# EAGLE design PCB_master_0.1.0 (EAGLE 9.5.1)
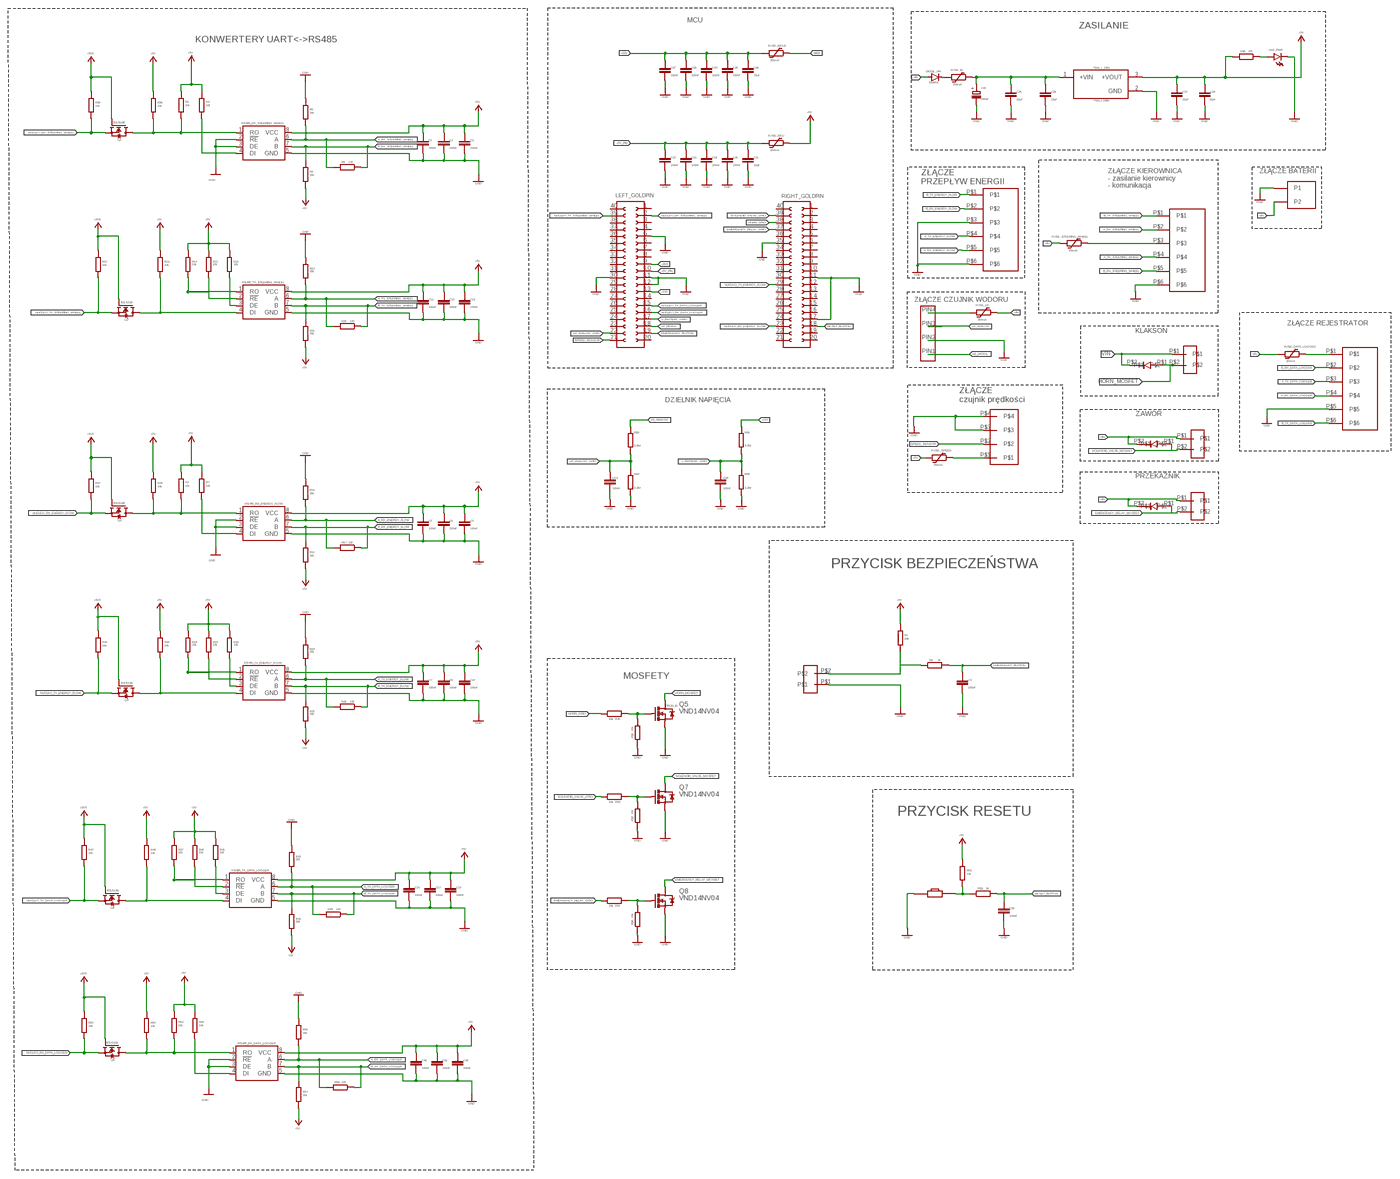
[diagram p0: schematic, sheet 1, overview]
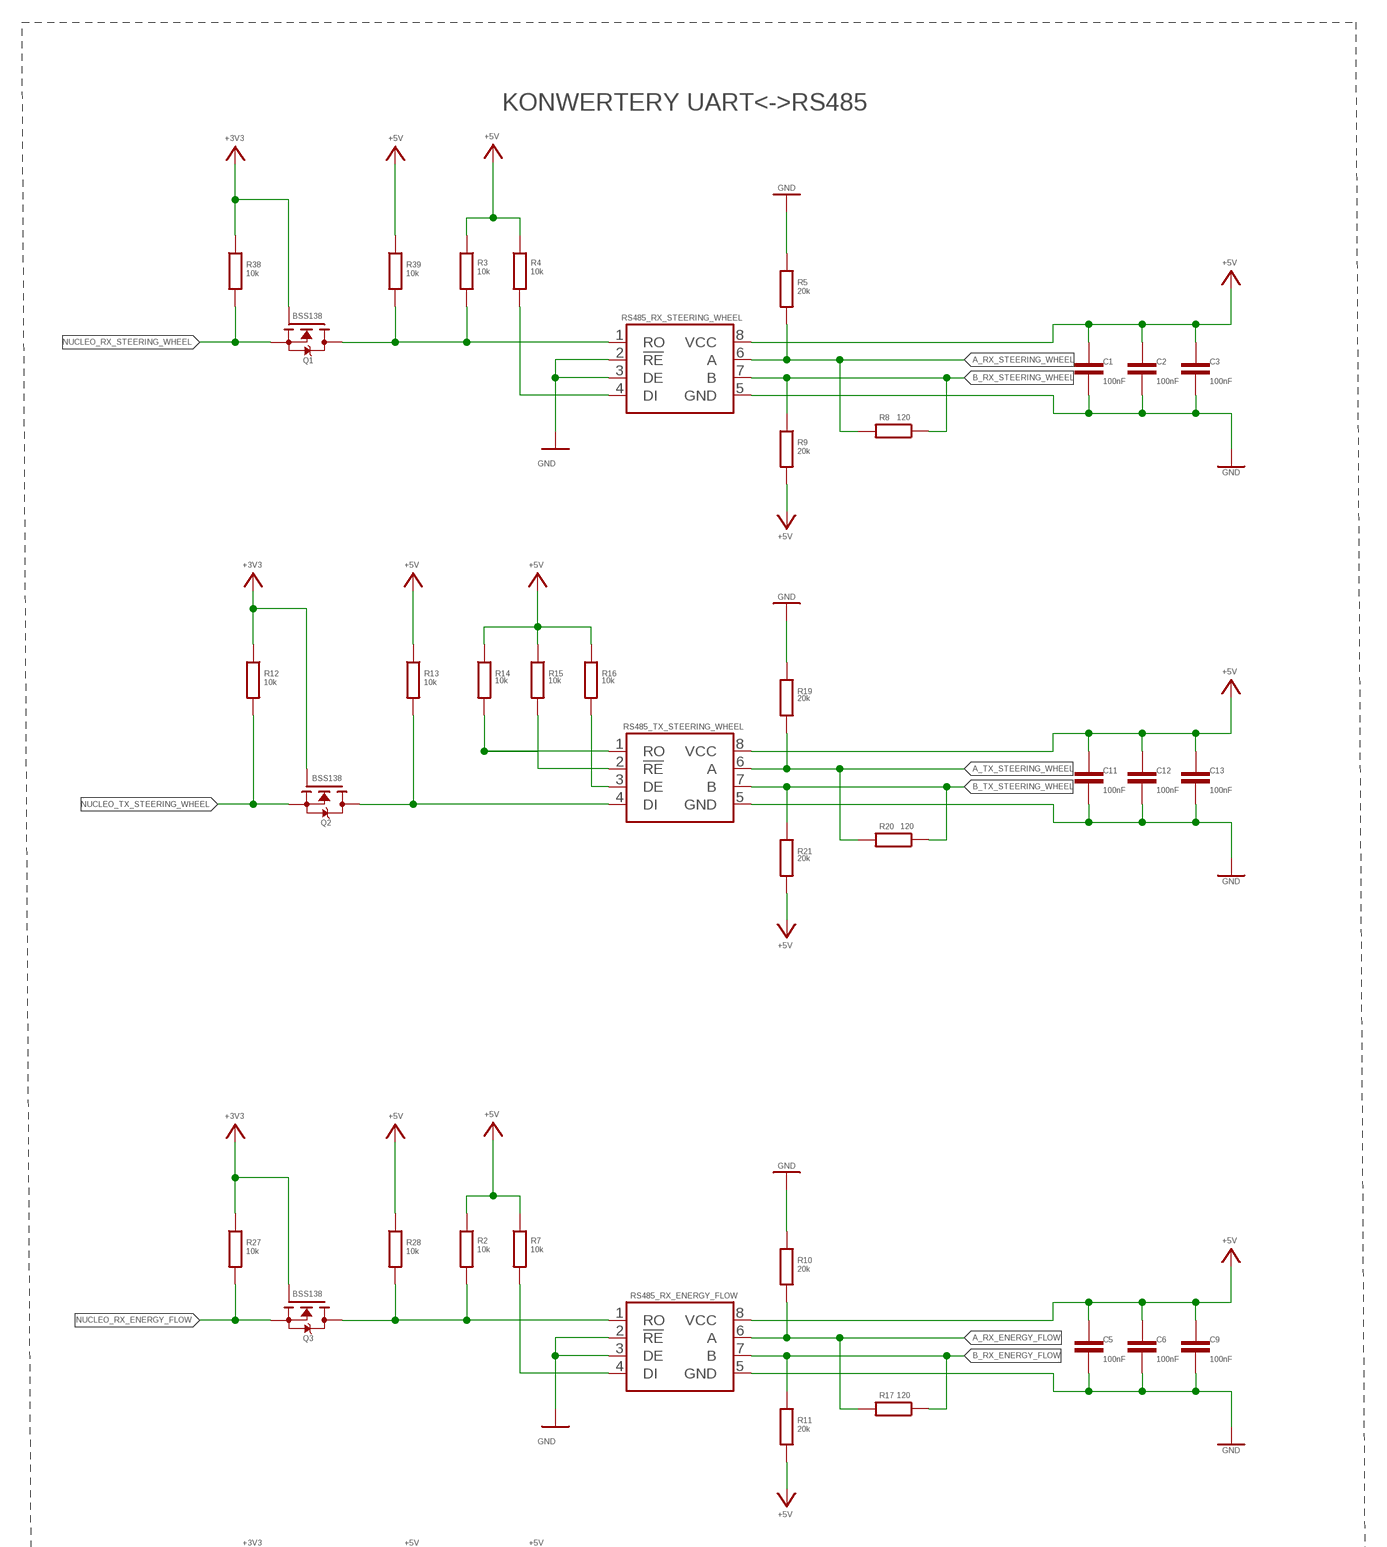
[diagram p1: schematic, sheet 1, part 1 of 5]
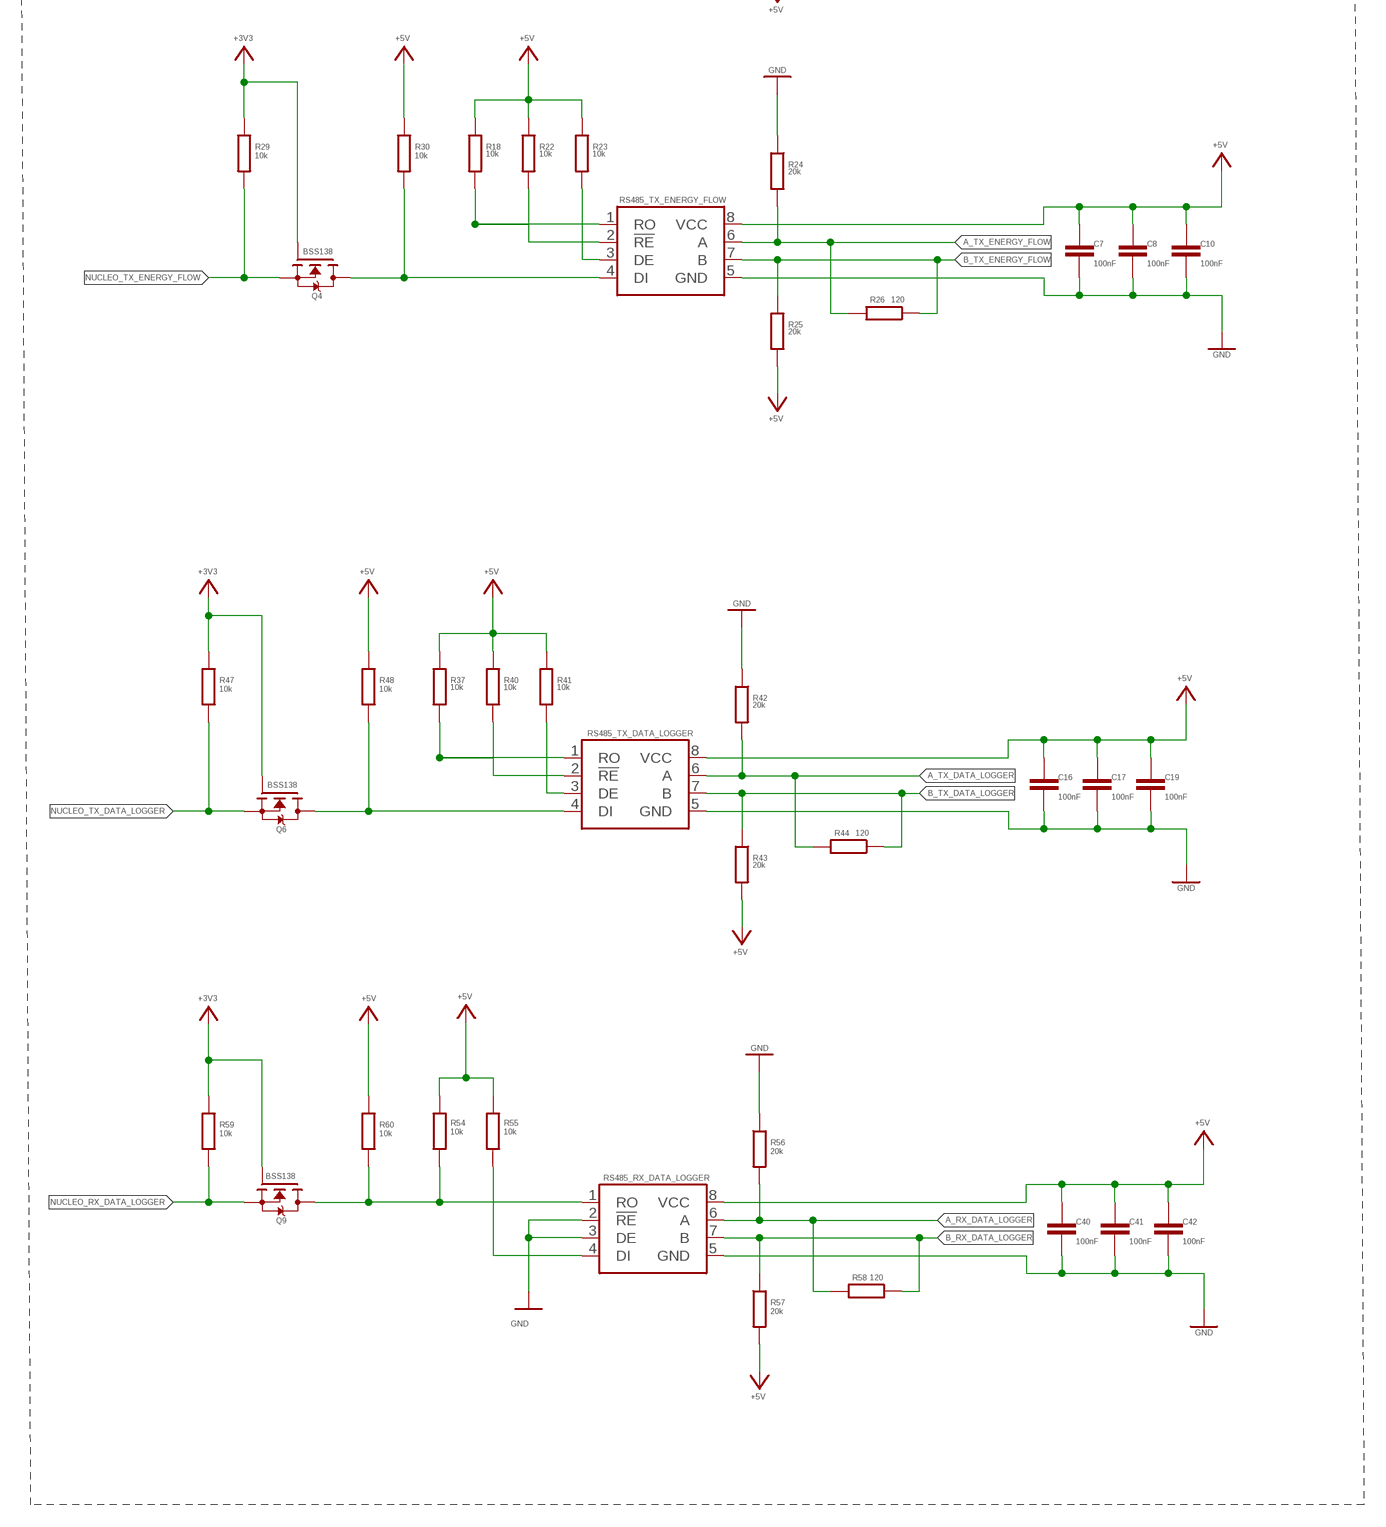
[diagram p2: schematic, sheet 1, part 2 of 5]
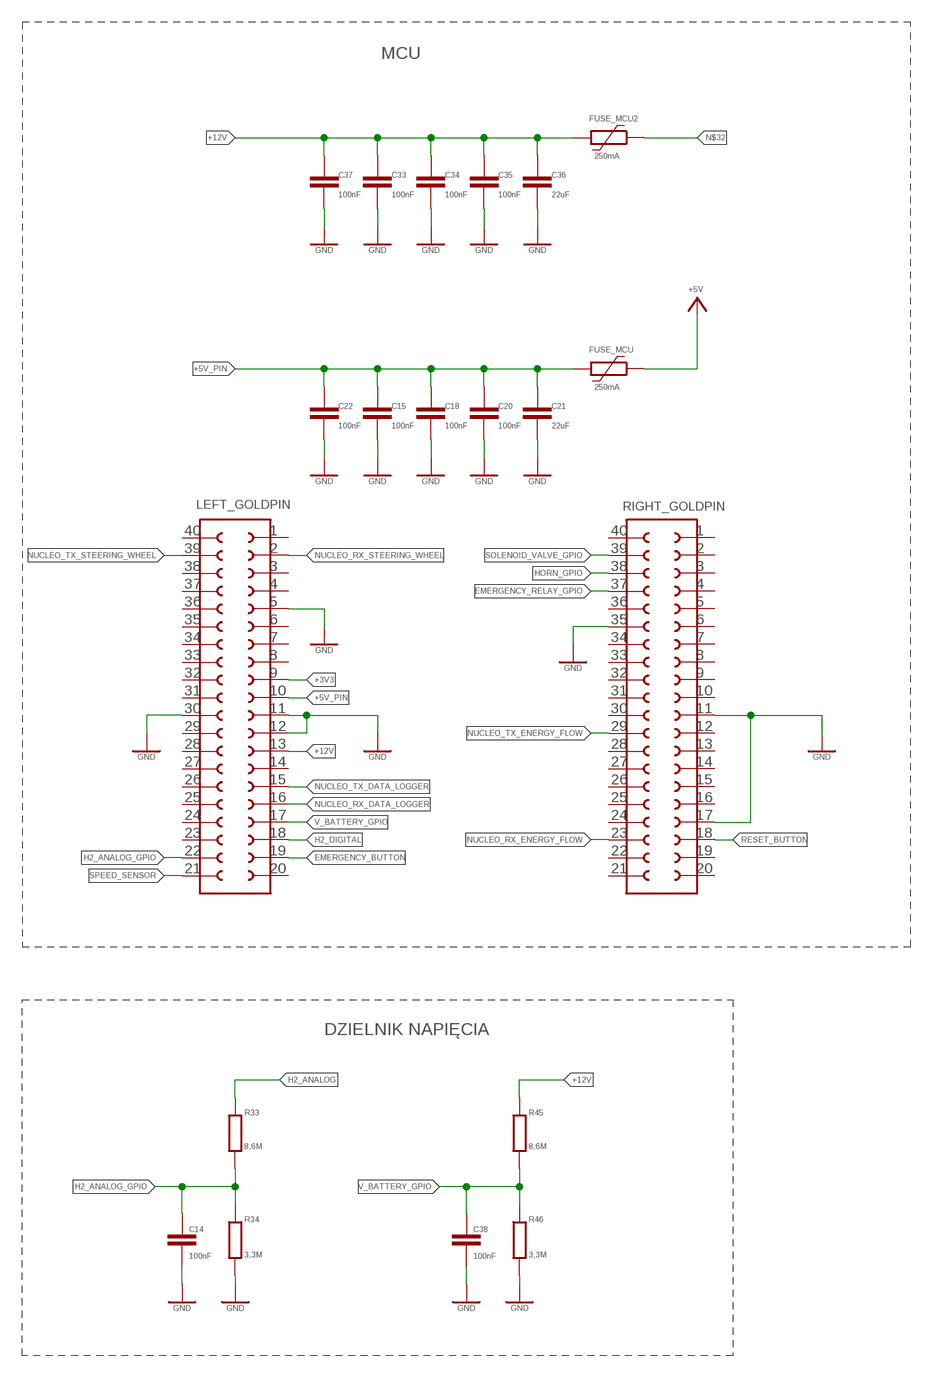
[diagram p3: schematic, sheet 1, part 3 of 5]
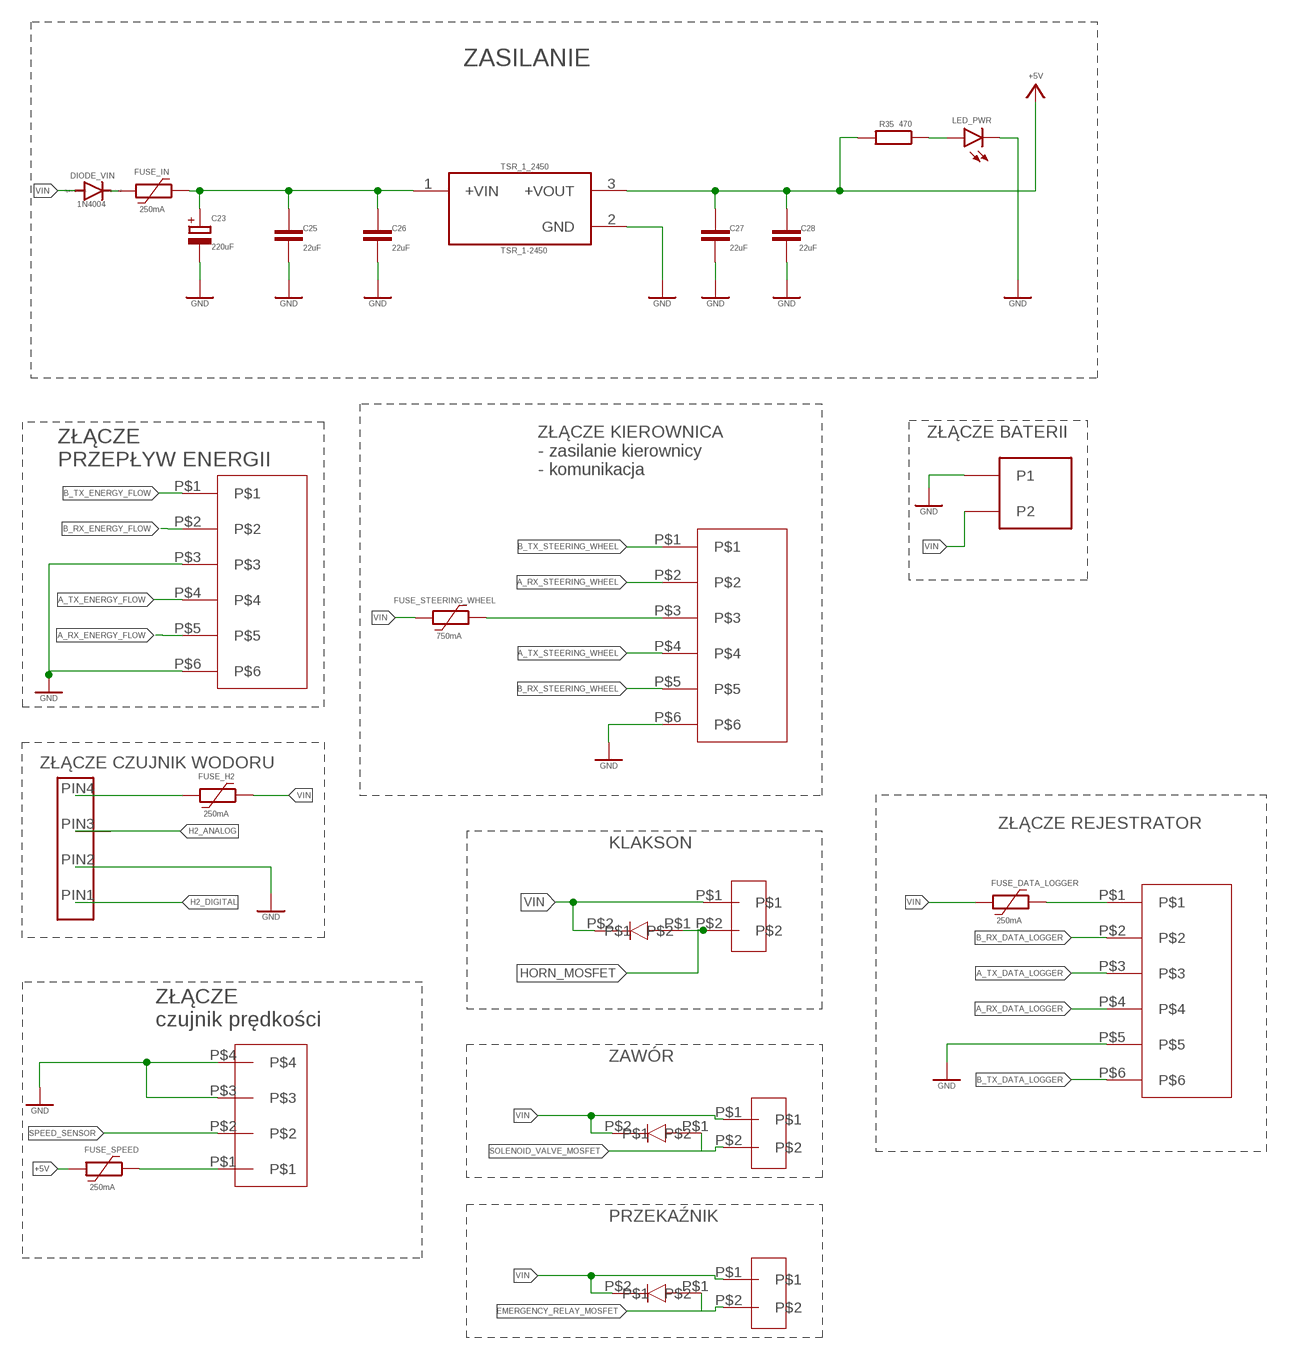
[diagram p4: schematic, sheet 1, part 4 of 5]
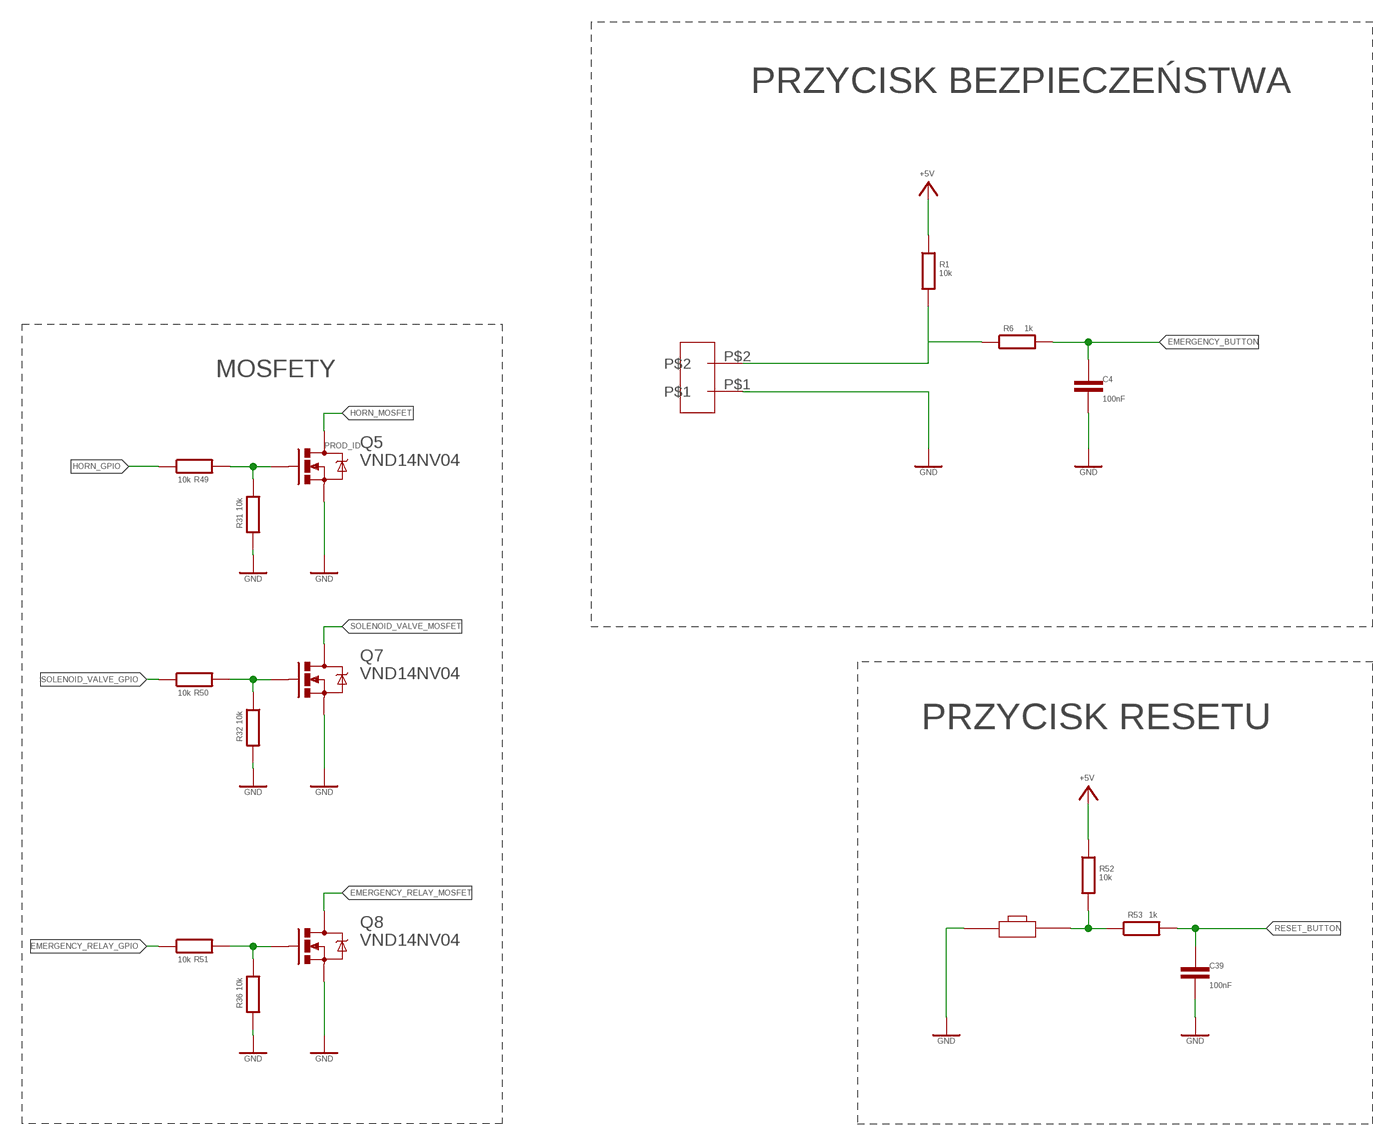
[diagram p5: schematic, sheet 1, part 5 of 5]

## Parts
C1  100nF  C-EUC1206  [C1206]
C2  100nF  C-EUC1206  [C1206]
C3  100nF  C-EUC1206  [C1206]
C4  100nF  C-EUC1206  [C1206]
C5  100nF  C-EUC1206  [C1206]
C6  100nF  C-EUC1206  [C1206]
C7  100nF  C-EUC1206  [C1206]
C8  100nF  C-EUC1206  [C1206]
C9  100nF  C-EUC1206  [C1206]
C10  100nF  C-EUC1206  [C1206]
C11  100nF  C-EUC1206  [C1206]
C12  100nF  C-EUC1206  [C1206]
C13  100nF  C-EUC1206  [C1206]
C14  100nF  C-EUC1206  [C1206]
C15  100nF  C-EUC1206  [C1206]
C16  100nF  C-EUC1206  [C1206]
C17  100nF  C-EUC1206  [C1206]
C18  100nF  C-EUC1206  [C1206]
C19  100nF  C-EUC1206  [C1206]
C20  100nF  C-EUC1206  [C1206]
C21  22uF  C-EUC1206  [C1206]
C22  100nF  C-EUC1206  [C1206]
C23  220uF  CPOL-EUUD-8X10  [UD-8X10_NICHICON]
C25  22uF  C-EUC1206  [C1206]
C26  22uF  C-EUC1206  [C1206]
C27  22uF  C-EUC1206  [C1206]
C28  22uF  C-EUC1206  [C1206]
C33  100nF  C-EUC1206  [C1206]
C34  100nF  C-EUC1206  [C1206]
C35  100nF  C-EUC1206  [C1206]
C36  22uF  C-EUC1206  [C1206]
C37  100nF  C-EUC1206  [C1206]
C38  100nF  C-EUC1206  [C1206]
C39  100nF  C-EUC1206  [C1206]
C40  100nF  C-EUC1206  [C1206]
C41  100nF  C-EUC1206  [C1206]
C42  100nF  C-EUC1206  [C1206]
DIODE_VIN  1N4004  [DO41-10]
FUSE_DATA_LOGGER  250mA  1206L012  [1206L]
FUSE_H2  250mA  1206L012  [1206L]
FUSE_IN  250mA  1206L012  [1206L]
FUSE_MCU  250mA  1206L012  [1206L]
FUSE_MCU2  250mA  1206L012  [1206L]
FUSE_SPEED  250mA  1206L012  [1206L]
FUSE_STEERING_WHEEL  750mA  2920L030  [2920L]
LED_PWR  LEDSMT1206  [1206]
LEFT_GOLDPIN  61304021821  [61304021821]
Q1  BSS138  [SOT23]
Q2  BSS138  [SOT23]
Q3  BSS138  [SOT23]
Q4  BSS138  [SOT23]
Q5  VND14NV04  MOSFET-NCHANNELFDD8780  [DPAK]
Q6  BSS138  [SOT23]
Q7  VND14NV04  MOSFET-NCHANNELFDD8780  [DPAK]
Q8  VND14NV04  MOSFET-NCHANNELFDD8780  [DPAK]
Q9  BSS138  [SOT23]
R1  10k  R-EU_R1206  [R1206]
R2  10k  R-EU_R1206  [R1206]
R3  10k  R-EU_R1206  [R1206]
R4  10k  R-EU_R1206  [R1206]
R5  20k  R-EU_R1206  [R1206]
R6  1k  R-EU_R1206  [R1206]
R7  10k  R-EU_R1206  [R1206]
R8  120  R-EU_R1206  [R1206]
R9  20k  R-EU_R1206  [R1206]
R10  20k  R-EU_R1206  [R1206]
R11  20k  R-EU_R1206  [R1206]
R12  10k  R-EU_R1206  [R1206]
R13  10k  R-EU_R1206  [R1206]
R14  10k  R-EU_R1206  [R1206]
R15  10k  R-EU_R1206  [R1206]
R16  10k  R-EU_R1206  [R1206]
R17  120  R-EU_R1206  [R1206]
R18  10k  R-EU_R1206  [R1206]
R19  20k  R-EU_R1206  [R1206]
R20  120  R-EU_R1206  [R1206]
R21  20k  R-EU_R1206  [R1206]
R22  10k  R-EU_R1206  [R1206]
R23  10k  R-EU_R1206  [R1206]
R24  20k  R-EU_R1206  [R1206]
R25  20k  R-EU_R1206  [R1206]
R26  120  R-EU_R1206  [R1206]
R27  10k  R-EU_R1206  [R1206]
R28  10k  R-EU_R1206  [R1206]
R29  10k  R-EU_R1206  [R1206]
R30  10k  R-EU_R1206  [R1206]
R31  10k  R-EU_R1206  [R1206]
R32  10k  R-EU_R1206  [R1206]
R33  8,2M  R-EU_M1206  [M1206]
R34  3,3M  R-EU_M1206  [M1206]
R35  470  R-EU_R1206  [R1206]
R36  10k  R-EU_R1206  [R1206]
R37  10k  R-EU_R1206  [R1206]
R38  10k  R-EU_R1206  [R1206]
R39  10k  R-EU_R1206  [R1206]
R40  10k  R-EU_R1206  [R1206]
R41  10k  R-EU_R1206  [R1206]
R42  20k  R-EU_R1206  [R1206]
R43  20k  R-EU_R1206  [R1206]
R44  120  R-EU_R1206  [R1206]
R45  8,7M  R-EU_M1206  [M1206]
R46  3,3M  R-EU_M1206  [M1206]
R47  10k  R-EU_R1206  [R1206]
R48  10k  R-EU_R1206  [R1206]
R49  10k  R-EU_R1206  [R1206]
R50  10k  R-EU_R1206  [R1206]
R51  10k  R-EU_R1206  [R1206]
R52  10k  R-EU_R1206  [R1206]
R53  1k  R-EU_R1206  [R1206]
R54  10k  R-EU_R1206  [R1206]
R55  10k  R-EU_R1206  [R1206]
R56  20k  R-EU_R1206  [R1206]
R57  20k  R-EU_R1206  [R1206]
R58  120  R-EU_R1206  [R1206]
R59  10k  R-EU_R1206  [R1206]
R60  10k  R-EU_R1206  [R1206]
RIGHT_GOLDPIN  61304021821  [61304021821]
RS485_RX_DATA_LOGGER  LTC485S  [SOIC8]
RS485_RX_ENERGY_FLOW  LTC485S  [SOIC8]
RS485_RX_STEERING_WHEEL  LTC485S  [SOIC8]
RS485_TX_DATA_LOGGER  LTC485S  [SOIC8]
RS485_TX_ENERGY_FLOW  LTC485S  [SOIC8]
RS485_TX_STEERING_WHEEL  LTC485S  [SOIC8]
TSR_1_2450  TSR_1-2450  [CONV_TSR_1-2450]
U$1  MOLEX_2PIN_KATOWY  [MOLEX_2PIN_KATOWY]
U$2  DO41_10_V  [D041_10_V]
U$3  DO41_10_V  [D041_10_V]
U$4  MOLEX_2PIN_KATOWY  [MOLEX_2PIN_KATOWY]
U$5  GNIAZDO_MOLEX_4PIN  [GNIAZDO_MOLEX_4PIN]
U$6  MOLEX_6PIN  [MOLEX_6PIN]
U$7  MOLEX_6PIN  [MOLEX_6PIN]
U$8  TACT_SWITCH  [TACT_SWITCH]
U$9  JST-4-PIN-ANGLE  [JST-4-PIN-ANGLE]
U$10  MOLEX_2PIN_KATOWY  [MOLEX_2PIN_KATOWY]
U$11  DO41_10_V  [D041_10_V]
U$13  MOLEX_2PIN_KATOWY  [MOLEX_2PIN_KATOWY]
U$14  MOLEX_6PIN  [MOLEX_6PIN]
U$15  XT-30F  [XT-30F]

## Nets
+3V3: LEFT_GOLDPIN.9 Q1.1(G) Q2.1(G) Q3.1(G) Q4.1(G) Q6.1(G) Q9.1(G) R12.1 R27.1 R29.1 R38.1 R47.1 R59.1
+5V: C1.2 C2.2 C3.2 C5.2 C6.2 C7.2 C8.2 C9.2 C10.2 C11.2 C12.2 C13.2 C16.2 C17.2 C19.2 C27.2 C28.2 C40.2 C41.2 C42.2 FUSE_MCU.1 FUSE_SPEED.2 R1.1 R2.1 R3.1 R4.1 R7.1 R9.2 R11.2 R13.1 R14.1 R15.1 R16.1 R18.1 R21.2 R22.1 R23.1 R25.2 R28.1 R30.1 R35.2 R37.1 R39.1 R40.1 R41.1 R43.2 R48.1 R52.1 R54.1 R55.1 R57.2 R60.1 RS485_RX_DATA_LOGGER.8(VCC) RS485_RX_ENERGY_FLOW.8(VCC) RS485_RX_STEERING_WHEEL.8(VCC) RS485_TX_DATA_LOGGER.8(VCC) RS485_TX_ENERGY_FLOW.8(VCC) RS485_TX_STEERING_WHEEL.8(VCC) TSR_1_2450.3(+VOUT)
+5V_PIN: C15.2 C18.2 C20.2 C21.2 C22.2 FUSE_MCU.2 LEFT_GOLDPIN.10
+12V: C33.2 C34.2 C35.2 C36.2 C37.2 FUSE_MCU2.2 LEFT_GOLDPIN.13 R45.2
A_RX_DATA_LOGGER: R56.2 R58.2 RS485_RX_DATA_LOGGER.6(A) U$14.P$4
A_RX_ENERGY_FLOW: R10.2 R17.2 RS485_RX_ENERGY_FLOW.6(A) U$7.P$5
A_RX_STEERING_WHEEL: R5.2 R8.2 RS485_RX_STEERING_WHEEL.6(A) U$6.P$2
A_TX_DATA_LOGGER: R42.2 R44.2 RS485_TX_DATA_LOGGER.6(A) U$14.P$3
A_TX_ENERGY_FLOW: R24.2 R26.2 RS485_TX_ENERGY_FLOW.6(A) U$7.P$4
A_TX_STEERING_WHEEL: R19.2 R20.2 RS485_TX_STEERING_WHEEL.6(A) U$6.P$4
B_RX_DATA_LOGGER: R57.1 R58.1 RS485_RX_DATA_LOGGER.7(B) U$14.P$2
B_RX_ENERGY_FLOW: R11.1 R17.1 RS485_RX_ENERGY_FLOW.7(B) U$7.P$2
B_RX_STEERING_WHEEL: R8.1 R9.1 RS485_RX_STEERING_WHEEL.7(B) U$6.P$5
B_TX_DATA_LOGGER: R43.1 R44.1 RS485_TX_DATA_LOGGER.7(B) U$14.P$6
B_TX_ENERGY_FLOW: R25.1 R26.1 RS485_TX_ENERGY_FLOW.7(B) U$7.P$1
B_TX_STEERING_WHEEL: R20.1 R21.1 RS485_TX_STEERING_WHEEL.7(B) U$6.P$1
EMERGENCY_BUTTON: C4.2 LEFT_GOLDPIN.19 R6.2
EMERGENCY_RELAY_GPIO: Q8.1(G) R36.1 R51.1 R51.2 RIGHT_GOLDPIN.37
EMERGENCY_RELAY_MOSFET: Q8.4(D) U$3.P$1 U$4.P$2
GND: C1.1 C2.1 C3.1 C4.1 C5.1 C6.1 C7.1 C8.1 C9.1 C10.1 C11.1 C12.1 C13.1 C14.1 C15.1 C16.1 C17.1 C18.1 C19.1 C20.1 C21.1 C22.1 C23.- C25.1 C26.1 C27.1 C28.1 C33.1 C34.1 C35.1 C36.1 C37.1 C38.1 C39.1 C40.1 C41.1 C42.1 LED_PWR.C LEFT_GOLDPIN.5 LEFT_GOLDPIN.11 LEFT_GOLDPIN.12 LEFT_GOLDPIN.30 Q5.3(S) Q7.3(S) Q8.3(S) R5.1 R10.1 R19.1 R24.1 R31.2 R32.2 R34.2 R36.2 R42.1 R46.2 R56.1 RIGHT_GOLDPIN.11 RIGHT_GOLDPIN.17 RIGHT_GOLDPIN.35 RS485_RX_DATA_LOGGER.2(!RE) RS485_RX_DATA_LOGGER.3(DE) RS485_RX_DATA_LOGGER.5(GND) RS485_RX_ENERGY_FLOW.2(!RE) RS485_RX_ENERGY_FLOW.3(DE) RS485_RX_ENERGY_FLOW.5(GND) RS485_RX_STEERING_WHEEL.2(!RE) RS485_RX_STEERING_WHEEL.3(DE) RS485_RX_STEERING_WHEEL.5(GND) RS485_TX_DATA_LOGGER.5(GND) RS485_TX_ENERGY_FLOW.5(GND) RS485_TX_STEERING_WHEEL.5(GND) TSR_1_2450.2(GND) U$5.P$3 U$5.P$4 U$6.P$6 U$7.P$3 U$7.P$6 U$8.P$1 U$9.PIN2 U$13.P$1 U$14.P$5 U$15.P1
H2_ANALOG: R33.2 U$9.PIN3
H2_ANALOG_GPIO: C14.2 LEFT_GOLDPIN.22 R33.1 R34.1
H2_DIGITAL: LEFT_GOLDPIN.18 U$9.PIN1
HORN_GPIO: Q5.1(G) R31.1 R49.1 R49.2 RIGHT_GOLDPIN.38
HORN_MOSFET: Q5.4(D) U$10.P$2 U$11.P$1
N$1: Q3.3(D) R2.2 R28.2 RS485_RX_ENERGY_FLOW.1(RO)
N$2: R7.2 RS485_RX_ENERGY_FLOW.4(DI)
N$3: R18.2 RS485_TX_ENERGY_FLOW.1(RO)
N$4: R22.2 RS485_TX_ENERGY_FLOW.2(!RE)
N$5: R23.2 RS485_TX_ENERGY_FLOW.3(DE)
N$6: Q4.3(D) R30.2 RS485_TX_ENERGY_FLOW.4(DI)
N$8: FUSE_SPEED.1 U$5.P$1
N$9: R37.2 RS485_TX_DATA_LOGGER.1(RO)
N$10: R40.2 RS485_TX_DATA_LOGGER.2(!RE)
N$11: R1.2 R6.1 U$13.P$2
N$12: R41.2 RS485_TX_DATA_LOGGER.3(DE)
N$13: Q6.3(D) R48.2 RS485_TX_DATA_LOGGER.4(DI)
N$14: FUSE_H2.2 U$9.PIN4
N$15: FUSE_STEERING_WHEEL.1 U$6.P$3
N$16: Q1.3(D) R3.2 R39.2 RS485_RX_STEERING_WHEEL.1(RO)
N$17: R4.2 RS485_RX_STEERING_WHEEL.4(DI)
N$18: R14.2 RS485_TX_STEERING_WHEEL.1(RO)
N$19: R15.2 RS485_TX_STEERING_WHEEL.2(!RE)
N$20: R16.2 RS485_TX_STEERING_WHEEL.3(DE)
N$21: Q2.3(D) R13.2 RS485_TX_STEERING_WHEEL.4(DI)
N$22: DIODE_VIN.C FUSE_IN.2
N$23: Q7.1(G) R32.1 R50.2
N$24: R52.2 R53.1 U$8.P$2
N$25: Q9.3(D) R54.2 R60.2 RS485_RX_DATA_LOGGER.1(RO)
N$26: R55.2 RS485_RX_DATA_LOGGER.4(DI)
N$28: LED_PWR.A R35.1
N$32: C23.+ C25.2 C26.2 FUSE_IN.1 FUSE_MCU2.1 TSR_1_2450.1(+VIN)
NUCLEO_RX_DATA_LOGGER: LEFT_GOLDPIN.16 Q9.2(S) R59.2
NUCLEO_RX_ENERGY_FLOW: Q3.2(S) R27.2 RIGHT_GOLDPIN.23
NUCLEO_RX_STEERING_WHEEL: LEFT_GOLDPIN.2 Q1.2(S) R38.2
NUCLEO_TX_DATA_LOGGER: LEFT_GOLDPIN.15 Q6.2(S) R47.2
NUCLEO_TX_ENERGY_FLOW: Q4.2(S) R29.2 RIGHT_GOLDPIN.29
NUCLEO_TX_STEERING_WHEEL: LEFT_GOLDPIN.39 Q2.2(S) R12.2
P$1: FUSE_DATA_LOGGER.1 U$14.P$1
RESET_BUTTON: C39.2 R53.2 RIGHT_GOLDPIN.18
SOLENOID_VALVE_GPIO: R50.1 RIGHT_GOLDPIN.39
SOLENOID_VALVE_MOSFET: Q7.4(D) U$1.P$2 U$2.P$1
SPEED_SENSOR: LEFT_GOLDPIN.21 U$5.P$2
V_BATTERY_GPIO: C38.2 LEFT_GOLDPIN.17 R45.1 R46.1
VIN: DIODE_VIN.A FUSE_DATA_LOGGER.2 FUSE_H2.1 FUSE_STEERING_WHEEL.2 U$1.P$1 U$2.P$2 U$3.P$2 U$4.P$1 U$10.P$1 U$11.P$2 U$15.P2
Unconnected: LEFT_GOLDPIN.1 LEFT_GOLDPIN.3 LEFT_GOLDPIN.4 LEFT_GOLDPIN.6 LEFT_GOLDPIN.7 LEFT_GOLDPIN.8 LEFT_GOLDPIN.14 LEFT_GOLDPIN.20 LEFT_GOLDPIN.23 LEFT_GOLDPIN.24 LEFT_GOLDPIN.25 LEFT_GOLDPIN.26 LEFT_GOLDPIN.27 LEFT_GOLDPIN.28 LEFT_GOLDPIN.29 LEFT_GOLDPIN.31 LEFT_GOLDPIN.32 LEFT_GOLDPIN.33 LEFT_GOLDPIN.34 LEFT_GOLDPIN.35 LEFT_GOLDPIN.36 LEFT_GOLDPIN.37 LEFT_GOLDPIN.38 LEFT_GOLDPIN.40 RIGHT_GOLDPIN.1 RIGHT_GOLDPIN.2 RIGHT_GOLDPIN.3 RIGHT_GOLDPIN.4 RIGHT_GOLDPIN.5 RIGHT_GOLDPIN.6 RIGHT_GOLDPIN.7 RIGHT_GOLDPIN.8 RIGHT_GOLDPIN.9 RIGHT_GOLDPIN.10 RIGHT_GOLDPIN.12 RIGHT_GOLDPIN.13 RIGHT_GOLDPIN.14 RIGHT_GOLDPIN.15 RIGHT_GOLDPIN.16 RIGHT_GOLDPIN.19 RIGHT_GOLDPIN.20 RIGHT_GOLDPIN.21 RIGHT_GOLDPIN.22 RIGHT_GOLDPIN.24 RIGHT_GOLDPIN.25 RIGHT_GOLDPIN.26 RIGHT_GOLDPIN.27 RIGHT_GOLDPIN.28 RIGHT_GOLDPIN.30 RIGHT_GOLDPIN.31 RIGHT_GOLDPIN.32 RIGHT_GOLDPIN.33 RIGHT_GOLDPIN.34 RIGHT_GOLDPIN.36 RIGHT_GOLDPIN.40

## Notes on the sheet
- MCU
- ZASILANIE
- KONWERTERY UART<->RS485
- ZŁĄCZE BATERII
- ZŁĄCZE 
  PRZEPŁYW ENERGII
- ZŁĄCZE KIEROWNICA
  - zasilanie kierownicy
  - komunikacja
- ZŁĄCZE CZUJNIK WODORU
- ZŁĄCZE REJESTRATOR
- KLAKSON
- DZIELNIK NAPIĘCIA
- ZŁĄCZE
  czujnik prędkości
- ZAWÓR
- PRZEKAŹNIK
- PRZYCISK BEZPIECZEŃSTWA
- MOSFETY
- PRZYCISK RESETU

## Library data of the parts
C1-C22 C25-C28 C33-C42 = rcl:C-EU: CAPACITOR, European symbol; SPICEPREFIX: C
C23 = rcl:CPOL-EU: POLARIZED CAPACITOR, European symbol; SPICEPREFIX: C
DIODE_VIN = diode:1N4004: DIODE
FUSE_DATA_LOGGER FUSE_H2 FUSE_IN FUSE_MCU FUSE_MCU2 FUSE_SPEED = polyfuse-smd_10:?: Polyfuse Resettable PTC; MF: Littelfuse; MPN: 1206L012; OC_FARNELL: 1596988; OC_NEWARK: 05M2298
FUSE_STEERING_WHEEL = polyfuse-smd_10:?: Polyfuse Resettable PTC; MF: Littelfuse; MPN: 2920L030; OC_FARNELL: 1822222; OC_NEWARK: 18M4789
LED_PWR = led:LED: LED
LEFT_GOLDPIN RIGHT_GOLDPIN = Wurth_Elektronik_Electromechanic_Board_to_Board_Connectors_rev16a:61304021821: WR-PHD 2.54mm Dual Socket Header, 40 Pins =>Code : Con_BTB_SHD_2.54_2_61304021821 Details see: http://katalog.we-online.de/en/em/613_0xx_218_21 Created 2014-05-29, Karrer Zheng 2014 (C) Würth Elektronik
Q1-Q4 Q6 Q9 = bss138_10:BSS138: BSS138 N-Channel Logic Level Enhancement Mode Field Effect Transistor Source: http://www.fairchildsemi.com/datasheets/BS/BSS138.pdf; MF: Fairchild; MPN: BSS138; OC_FARNELL: 9845330; OC_NEWARK: 67R2009
Q5 Q7 Q8 = BeagleBone_Blue_R3:MOSFET-NCHANNEL: Common NMOSFET Parts MFG P/NStore IDProd ID FDD8780TRANS-09984 SI7820DNTRANS-11055 FDS6630AIC-08089 2N7002PWTRANS-11151 FQP30N06L COM-10213TRANS-10060 BSS123LT1GTRANS-08345 BSS138TRANS-00830 BS170 2N7000; PROD_ID: TRANS-09984
R1-R60 = rcl:R-EU_: RESISTOR, European symbol; SPICEPREFIX: R
RS485_RX_DATA_LOGGER RS485_RX_ENERGY_FLOW RS485_RX_STEERING_WHEEL RS485_TX_DATA_LOGGER RS485_TX_ENERGY_FLOW RS485_TX_STEERING_WHEEL = linear-technology:LTC485: Low Power RS485 Interface Transceiver Source: http://www.linear.com/pc/downloadDocument.do?navId=H0,C1,C1007,C1017,P2064,D1718; OC_FARNELL: unknown; OC_NEWARK: unknown
TSR_1_2450 = TSR_1-2450:TSR_1-2450: Linear Regulator Replacement DC DC Converter 1 Output 12V 1A 15V - 36V Input; AVAILABILITY: Unavailable; DESCRIPTION: Linear Regulator Replacement DC DC Converter 1 Output 5V 1A 6.5V - 36V Input; MF: Traco Power; MP: TSR 1-2450; PACKAGE: SIP-3 Tracopower; PRICE: None
U$1 U$4 U$10 U$13 = Molex_2pin_angle:MOLEX_2PIN_KATOWY
U$2 U$3 U$11 = DIODE_VERTICAL_DO41:DO41_10_V
U$5 = MOLEX_4PIN:GNIAZDO_MOLEX_4PIN
U$6 U$7 U$14 = MOLEX_6PIN:MOLEX_6PIN
U$8 = TACT_SWITCH:TACT_SWITCH
U$9 = PIN-ANGLE-mod:JST-4-PIN-ANGLE
U$15 = XT_30:XT-30F

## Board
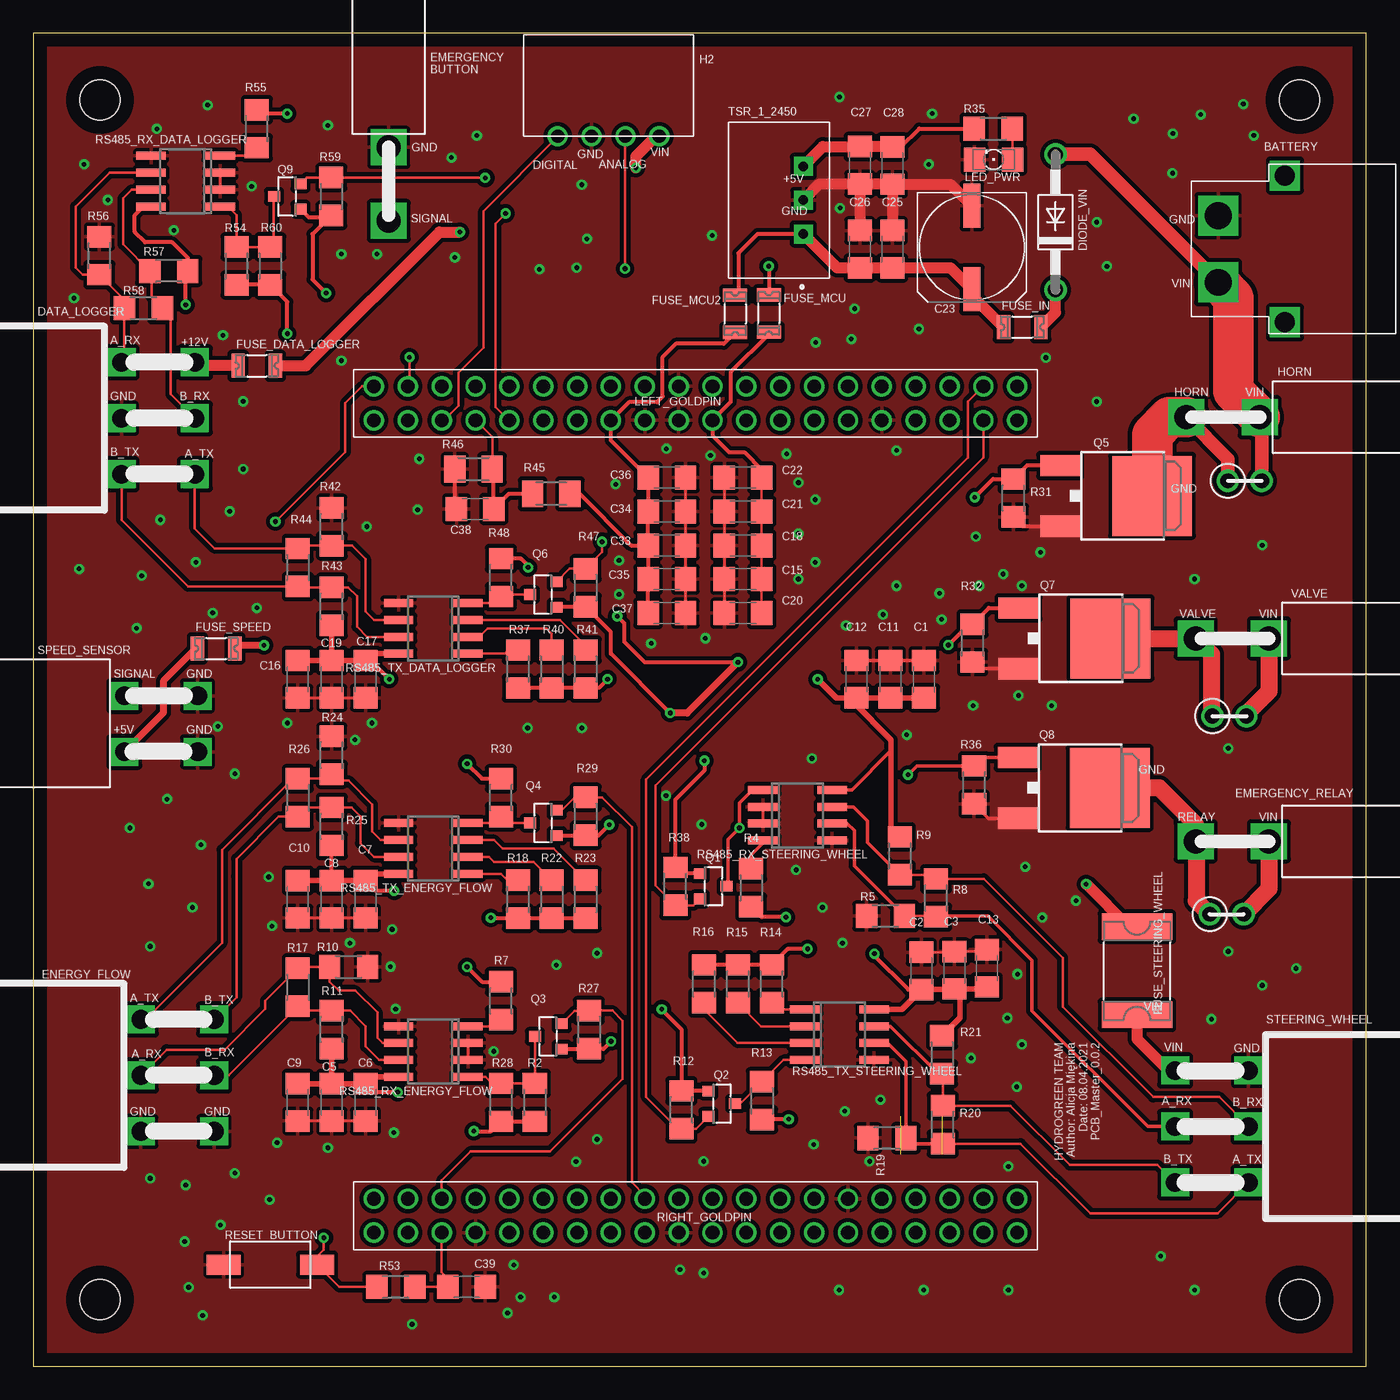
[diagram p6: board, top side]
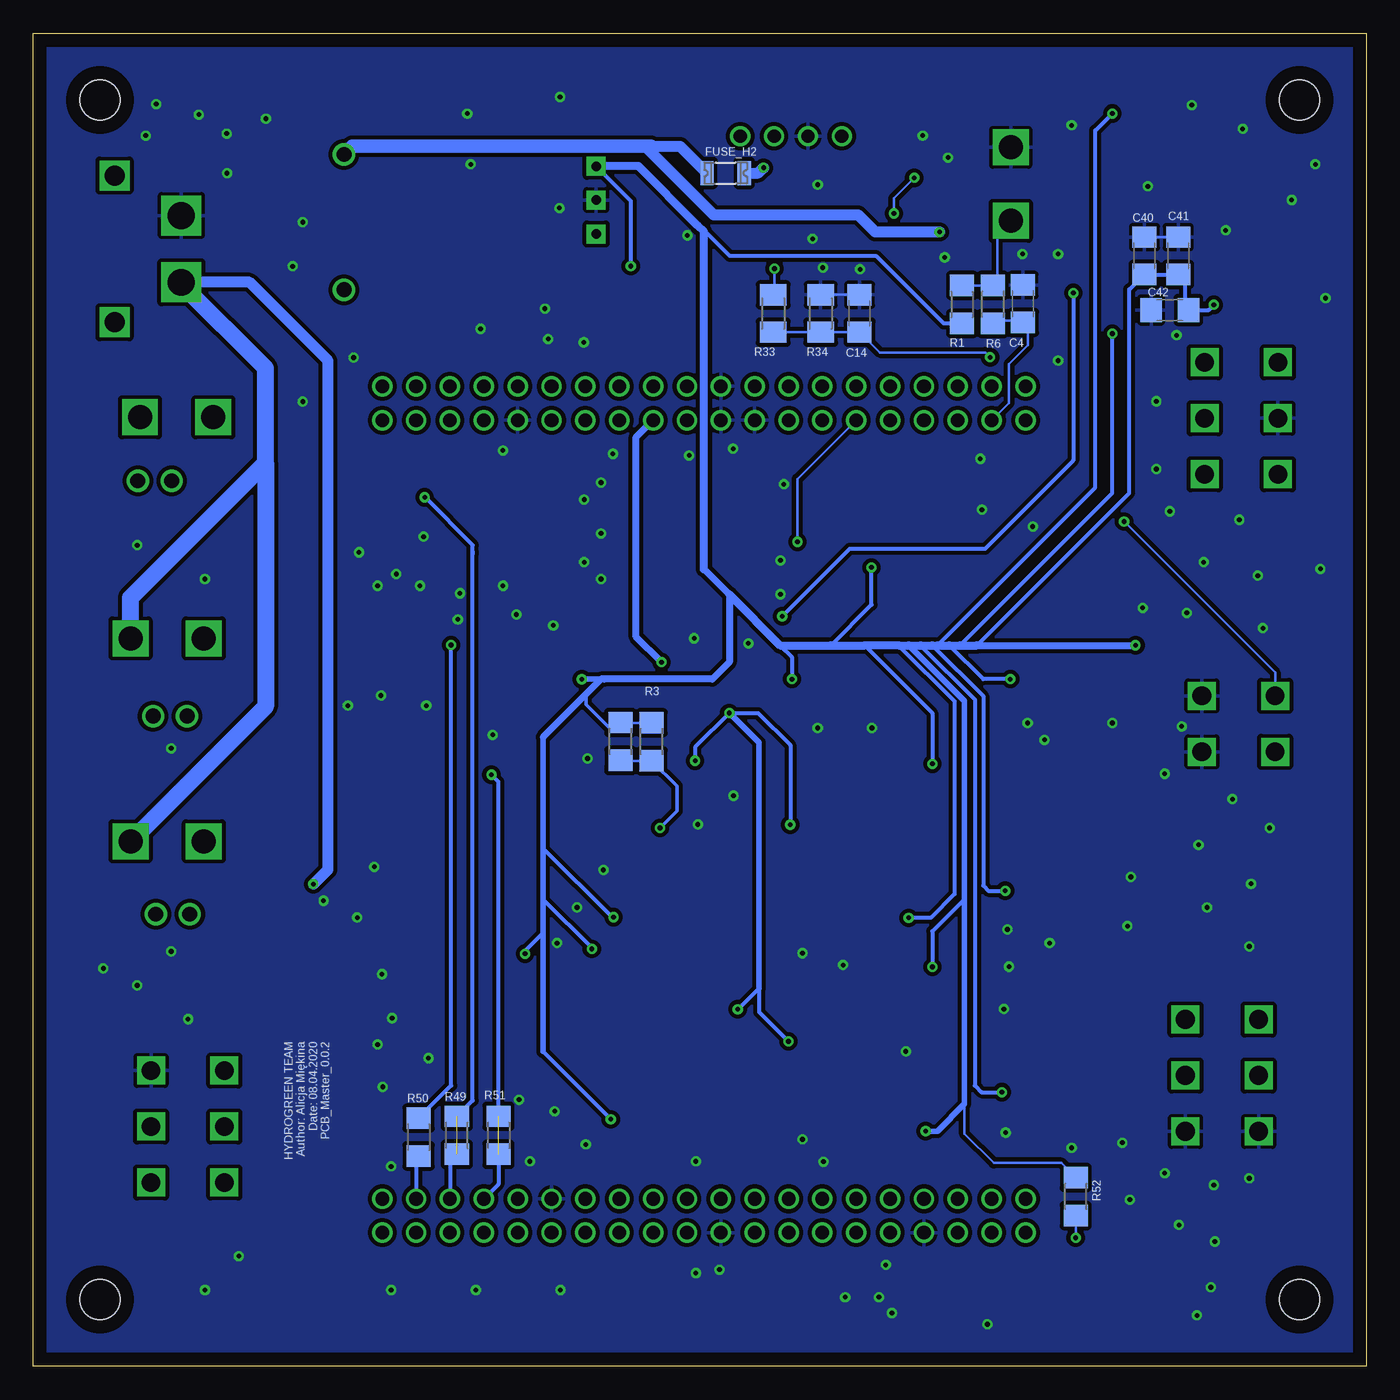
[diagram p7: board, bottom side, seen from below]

Size 100 x 100 mm. Coordinates in mm from the lower left corner, seen from the top.
Outline: 0,0 100,0 100,100 0,100 0,0
Copper layers (1*16): Top 0.035mm / dielectric 1.5mm / Bottom 0.035mm
Design rules "default *": minimum track width 6mil, minimum drill 0.35mm, track to track 6mil, track to pad 6mil, pad to pad 6mil, via to via 6mil, smd to smd 6mil, copper to edge 40mil, drill to drill 6mil, minimum pad ring 10mil, minimum via ring 8mil, stop-mask expansion 4mil, vias tented up to drill 0mil, thermal gap 10mil
Holes 3 mm at 5,5 5,95 95,95 95,5

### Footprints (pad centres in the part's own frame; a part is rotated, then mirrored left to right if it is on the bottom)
C1206 = smd 1.6 x 1.8: 1 -1.4,0; 2 1.4,0
UD-8X10_NICHICON = smd 3.3 x 1.3: + 3.125,0; - -3.125,0
DO41-10 = drill 1.118: A 5.08,0; C -5.08,0
1206L = smd 1 x 1.8: 1 -1.4,0; 2 1.4,0
2920L = smd 2 x 5.3: 1 -3.3,0; 2 3.3,0
1206 = smd 1.6 x 1.803: A -1.422,0; C 1.422,0
61304021821 = drill 1.02: 1 -24.13,1.27; 2 -21.59,1.27; 3 -19.05,1.27; 4 -16.51,1.27; 5 -13.97,1.27; 6 -11.43,1.27; 7 -8.89,1.27; 8 -6.35,1.27; 9 -3.81,1.27; 10 -1.27,1.27; 11 1.27,1.27; 12 3.81,1.27; 13 6.35,1.27; 14 8.89,1.27; 15 11.43,1.27; 16 13.97,1.27; 17 16.51,1.27; 18 19.05,1.27; 19 21.59,1.27; 20 24.13,1.27; 21 24.13,-1.27; 22 21.59,-1.27; 23 19.05,-1.27; 24 16.51,-1.27; 25 13.97,-1.27; 26 11.43,-1.27; 27 8.89,-1.27; 28 6.35,-1.27; 29 3.81,-1.27; 30 1.27,-1.27; 31 -1.27,-1.27; 32 -3.81,-1.27; 33 -6.35,-1.27; 34 -8.89,-1.27; 35 -11.43,-1.27; 36 -13.97,-1.27; 37 -16.51,-1.27; 38 -19.05,-1.27; 39 -21.59,-1.27; 40 -24.13,-1.27
SOT23 = smd 0.8 x 0.9: 1 -0.95,-1; 2 0.95,-1; 3 0,1
DPAK = smd 1.6 x 2.997: 1 -2.28,-5.31; 3 2.28,-5.31 | smd 5.994 x 5.994: 4 0,1.588
R1206 = smd 1.6 x 1.803: 1 -1.422,0; 2 1.422,0
M1206 = smd 1.6 x 2: 1 -1.4,0; 2 1.4,0
SOIC8 = smd 0.6 x 2.2: 1 -1.905,-2.6; 2 -0.635,-2.6; 3 0.635,-2.6; 4 1.905,-2.6; 5 1.905,2.6; 6 0.635,2.6; 7 -0.635,2.6; 8 -1.905,2.6
CONV_TSR_1-2450 = drill 0.71 pad 1.422 square: 1 -2.54,0; 2 0,0; 3 2.54,0
MOLEX_2PIN_KATOWY = drill 1.8 square: P$1 0,0; P$2 -5.5,0
D041_10_V = drill 1.118: P$1 -1.27,0; P$2 1.27,0
GNIAZDO_MOLEX_4PIN = drill 1.4 square: P$1 2.145,1.06; P$2 -2.055,1.06; P$3 -2.055,6.56; P$4 2.145,6.56
MOLEX_6PIN = drill 1.4 square: P$1 -4.196,5.517; P$2 0.004,5.517; P$3 4.204,5.517; P$4 -4.196,0.017; P$5 0.004,0.017; P$6 4.204,0.017
TACT_SWITCH = smd 2.54 x 1.5: P$1 3.5,0; P$2 -3.5,0
JST-4-PIN-ANGLE = drill 1: PIN1 -2.54,0; PIN2 0,0; PIN3 2.54,0; PIN4 5.08,0
XT-30F = drill 1.5 square: C1 -5.5,5; C2 5.5,5 | drill 2 square: P1 -2.5,0; P2 2.5,0

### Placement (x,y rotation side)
C1  66.83,51.55 270 top
C2  66.63,29.65 270 top
C3  69.12,29.7 270 top
C4  25.75,79.71 270 bottom
C5  22.38,19.8 90 top
C6  24.92,19.8 90 top
C7  24.92,35.04 90 top
C8  22.38,35.04 90 top
C9  19.84,19.8 90 top
C10  19.84,35.04 90 top
C11  64.29,51.55 270 top
C12  61.75,51.55 270 top
C13  71.53,29.85 270 top
C14  38.01,78.98 270 bottom
C15  53.24,59.04 0 top
C16  19.84,51.55 90 top
C17  24.92,51.55 90 top
C18  53.24,61.58 0 top
C19  22.38,51.55 90 top
C20  53.24,56.5 0 top
C21  53.24,64.12 0 top
C22  53.24,66.66 0 top
C23  70.42,83.93 270 top
C25  64.45,83.8 270 top
C26  62.01,83.8 270 top
C27  62.01,90.1 90 top
C28  64.45,90.08 90 top
C33  47.53,61.58 180 top
C34  47.53,64.12 180 top
C35  47.53,59.04 180 top
C36  47.53,66.66 180 top
C37  47.53,56.5 180 top
C38  33.15,64.31 0 top
C39  32.51,5.94 180 top
C40  16.64,83.31 270 bottom
C41  14.1,83.31 270 bottom
C42  14.73,79.25 0 bottom
DIODE_VIN  76.69,85.84 90 top
FUSE_DATA_LOGGER  16.76,75.06 0 top
FUSE_H2  48.06,89.51 0 bottom
FUSE_IN  74.19,77.95 0 top
FUSE_MCU  55.18,78.98 270 top
FUSE_MCU2  52.66,78.95 270 top
FUSE_SPEED  13.72,53.85 0 top
FUSE_STEERING_WHEEL  82.8,29.67 90 top
LED_PWR  72.04,90.53 180 top
LEFT_GOLDPIN  49.69,72.25 180 top
Q1  51.01,36 270 top
Q2  51.64,19.69 270 top
Q3  38.64,24.75 90 top
Q4  38.26,40.75 90 top
Q5  82.35,65.29 270 top
Q6  38.26,57.9 90 top
Q7  79.23,54.61 270 top
Q8  79.17,43.38 270 top
Q9  19.05,87.76 90 top
R1  30.32,79.66 90 bottom
R2  37.62,19.8 90 top
R3  53.61,46.85 270 bottom
R4  53.85,35.9 90 top
R5  63.94,33.77 0 top
R6  28.01,79.66 270 bottom
R7  35.08,27.42 270 top
R8  67.72,35.14 270 top
R9  65.01,38.29 90 top
R10  23.65,29.96 180 top
R11  22.38,25.26 270 top
R12  48.62,19.24 270 top
R13  54.67,19.92 90 top
R14  55.4,28.69 270 top
R15  52.86,28.69 270 top
R16  50.32,28.69 270 top
R17  19.84,28.43 90 top
R18  36.35,35.04 90 top
R19  64.04,17.11 0 top
R20  68.23,18.12 270 top
R21  68.18,23.38 90 top
R22  38.89,35.04 90 top
R23  41.43,35.04 90 top
R24  22.38,45.83 270 top
R25  22.38,40.5 270 top
R26  19.84,42.66 90 top
R27  41.69,25.26 90 top
R28  35.08,19.8 90 top
R29  41.43,41.26 90 top
R30  35.08,42.66 270 top
R31  73.54,65.14 270 top
R32  70.46,54.25 270 top
R33  44.48,78.98 90 bottom
R34  40.93,78.98 90 bottom
R35  72.02,92.85 180 top
R36  70.59,43.61 270 top
R37  36.35,52.31 90 top
R38  48.16,36 270 top
R39  55.95,46.87 270 bottom
R40  38.89,52.31 90 top
R41  41.43,52.31 90 top
R42  22.38,62.98 270 top
R43  22.38,57.01 270 top
R44  19.84,59.93 90 top
R45  38.86,65.46 0 top
R46  33.02,67.31 180 top
R47  41.43,58.4 90 top
R48  35.08,59.17 270 top
R49  68.22,17.32 270 bottom
R50  71.09,17.2 90 bottom
R51  65.1,17.32 90 bottom
R52  21.79,12.73 270 bottom
R53  27.2,5.94 0 top
R54  15.24,82.55 90 top
R55  16.76,92.84 270 top
R56  4.95,83.31 270 top
R57  10.16,82.17 0 top
R58  8.26,79.38 180 top
R59  22.35,87.76 90 top
R60  17.78,82.55 90 top
RIGHT_GOLDPIN  49.69,11.29 180 top
RS485_RX_DATA_LOGGER  11.43,88.9 90 top
RS485_RX_ENERGY_FLOW  30,23.61 90 top
RS485_RX_STEERING_WHEEL  57.33,41.34 270 top
RS485_TX_DATA_LOGGER  30,55.36 90 top
RS485_TX_ENERGY_FLOW  30,38.85 90 top
RS485_TX_STEERING_WHEEL  60.48,24.88 270 top
TSR_1_2450  57.77,87.49 90 top
U$1  92.71,54.61 0 top
U$2  89.74,48.77 0 top
U$3  89.53,33.91 0 top
U$4  92.71,39.37 0 top
U$5  5.77,48.23 270 top
U$6  91.19,17.98 90 top
U$7  8.05,21.82 270 top
U$8  17.78,7.62 180 top
U$9  41.88,92.28 0 top
U$10  92,71.19 0 top
U$11  90.89,66.43 0 top
U$13  26.67,91.44 90 top
U$14  6.6,71.12 270 top
U$15  88.9,83.82 270 top

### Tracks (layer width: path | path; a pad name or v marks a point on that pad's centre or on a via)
+3V3  (via drill 0.35)
  Top 0.305: Q1.1 48.64,36.95 R38.1 48.16,42.5 50.35,44.69 v50.35,45.42 | Q2.1 48.64,20.64 R12.1 48.62,25.28 47.15,26.75 v47.15,26.78 | Q4.1 41.4,39.8 | 41.4,39.8 R29.1 | Q3.1 41.65,23.8 | 41.65,23.8 R27.1 | Q6.1 41.4,56.95 R47.1 43.34,55.08 43.34,53.45 v47.78,49.01 | v43.21,40.62 42.39,39.8 41.4,39.8 | v43.34,24.37 42.77,23.8 41.65,23.8 | Q9.1 20.68,86.17 22.19,86.17 R59.1 20.95,84.94 20.95,81.53 v21.97,80.52 | v43.81,56.26 44.32,55.75 44.32,54.36 45.86,52.82 v52.86,52.82
  Top 0.508: v52.86,52.82 49.05,49.01 v47.78,49.01
  Bottom 0.305: v43.21,40.62 43.21,46.59 45.62,49.01 v47.78,49.01 50.35,46.44 v50.35,45.42 | v43.34,24.37 45.52,26.55 45.52,30.95 45.57,30.9 | 45.57,28.36 v47.15,26.78 | v43.81,56.26 38.73,61.34 28.57,61.34 21.97,67.94 v21.97,80.52
  Bottom 0.406: v47.78,49.01 45.57,46.8 45.57,30.9 45.57,28.36
  Bottom 0.508: v52.86,52.82 54.77,54.72 54.77,69.71 LEFT_GOLDPIN.9
+5V  (via drill 0.35)
  Top 0.254: RS485_RX_STEERING_WHEEL.8 61.42,43.24 64.35,46.18
  Top 0.305: C8.2 R25.2 | R23.1 R22.1 R18.1 36.33,33.64 v34.32,33.64 | R16.1 R15.1 R14.1 56.6,31.3 v58.1,31.3 | R37.1 R40.1 R41.1 42.42,50.89 v43.09,51.55 | C28.2 65.11,91.48 66.48,92.85 R35.2 | R2.1 R28.1 34.35,17.64 v33.05,17.64 | v26.7,51.55 25.3,52.95 C17.2 | v27.08,35.67 25.69,35.67 C7.2 | v27.34,20.56 25.56,20.56 C6.2 | R48.1 36.58,60.59 37.12,60.05 v37.12,59.93 | v32.54,45.2 33.66,44.08 R30.1 | v32.54,29.96 33.66,28.84 R7.1 | v56.67,18.53 56.65,18.5 R13.1 | R4.1 54.64,33.69 v56.47,33.69 | C2.2 65.64,28.25 63.02,30.87 v63.1,30.95 | v55.17,82.53 FUSE_MCU.1 | v11.43,79.63 11.43,82.02 R57.2 11.58,83.16 10.41,84.33 8.38,84.33 7.62,85.09 7.62,86.36 8.26,87 RS485_RX_DATA_LOGGER.8 | v19.05,77.47 19.05,79.86 R60.1 R54.1 | v19.05,93.98 17.04,93.98 R55.1
  Top 0.406: C1.2 C11.2 C12.2 61.52,50.15 | RS485_TX_STEERING_WHEEL.8 65.19,26.78 66.63,28.23 C2.2 69.07,28.25 C3.2 | C13.2 71.38,28.3 C3.2 | R21.2 69.53,26.15 69.53,27.9 C3.2 | RS485_TX_ENERGY_FLOW.8 25.43,36.94 C7.2 C8.2 C10.2 | RS485_RX_ENERGY_FLOW.8 25.43,21.7 C6.2 C5.2 | C9.2 C5.2 | C5.2 R11.2 | RS485_TX_DATA_LOGGER.8 25.43,53.45 C17.2 C19.2 | C19.2 C16.2 | C19.2 R43.2 | v58.85,51.54 60.24,50.15 61.52,50.15 | 61.52,50.15 61.52,49.83 64.35,46.99 64.35,46.18 64.35,40.36 R9.2
  Top 0.508: v17.3,54.09 15.35,54.09 FUSE_SPEED.2
  Top 0.813: TSR_1_2450.3 59.24,91.5 C27.2 62.03,91.48 C28.2
  Bottom 0.203: R39.1 55.92,48.27 R3.1 | R52.1 21.79,14.17 22.86,15.24 27.94,15.24 30.13,17.43 30.13,19.67
  Bottom 0.254: R39.1 56.57,47.68 58.52,49.63 58.52,50.44
  Bottom 0.305: TSR_1_2450.3 55.17,87.44 v55.17,82.53 | 31.27,54.09 28.73,51.55 v26.7,51.55 | 33.43,54.09 29.37,50.02 29.37,21.07 28.86,20.56 v27.34,20.56 | 35.08,54.09 30.89,49.9 30.89,35.42 32.67,33.64 v34.32,33.64 | v27.08,35.67 28.35,35.67 28.73,36.05 28.73,50.28 32.54,54.09 32.16,54.09 20.32,65.93 20.32,92.71 v19.05,93.98 | 43.97,54.09 43.09,53.2 v43.09,51.55 | 40.16,54.09 37.12,57.13 v37.12,59.93 | 37.62,54.09 32.54,49.01 v32.54,45.2 | 30.13,35.04 32.54,32.62 v32.54,29.96 | 55.99,48.57 R39.1 | 61.75,23.61 v56.67,18.53 | 61.75,38.85 56.6,33.69 v56.47,33.69 | 61.75,35.04 58.1,31.38 v58.1,31.3 | v63.1,30.95 63.1,31.15 61.75,32.5 | 50.15,85.59 50.03,85.59 47.75,83.31 36.79,83.31 31.72,78.24 R1.1 | 29.21,54.09 17.78,65.52 17.78,80.77 C40.2 C41.2 13.59,81.4 13.59,79.5 C42.2 11.81,79.25 v11.43,79.63 | 30.48,54.09 19.05,65.52 v19.05,77.47
  Bottom 0.406: 34.32,54.09 30.13,49.9 30.13,35.04 30.13,19.67 32.16,17.64 v33.05,17.64 | 61.75,47.2 61.75,38.85 61.75,35.04 61.75,32.5 61.75,23.61 | 57.15,51.55 v58.84,51.55 v58.85,51.54
  Bottom 0.508: 57.74,90.05 TSR_1_2450.3 | 49.69,59.8 47.78,57.9 47.78,52.82 49.05,51.55 57.15,51.55 57.41,51.55 58.52,50.44 61.75,47.2 | 29.21,54.09 v17.3,54.09
  Bottom 0.61: 57.74,90.05 54.62,90.05 50.15,85.59 49.69,85.12 49.69,59.8 | 47.78,57.9 43.97,54.09 40.16,54.09 37.62,54.09 35.08,54.09 34.32,54.09 33.43,54.09 32.54,54.09 30.48,54.09 29.21,54.09 | 32.16,54.09 31.27,54.09
+5V_PIN
  Top 0.203: C22.2 C21.2 C18.2 C15.2 C20.2
  Top 0.305: FUSE_MCU.2 55.17,77.43 52.32,74.57 52.32,72.34 LEFT_GOLDPIN.10 50.96,69.82 52.2,68.58 53.34,68.58 54.65,67.28 C22.2
+12V
  Top 0.305: C33.2 C34.2 C36.2 43.34,69.45 LEFT_GOLDPIN.13 44.69,72.33 46.8,72.33 47.22,72.75 47.22,75.72 48.21,76.71 51.82,76.71 FUSE_MCU2.2 | C33.2 C35.2 C37.2 | R45.2 40.98,65.46 44.86,61.58 C33.2
A_RX_DATA_LOGGER
  Top 0.203: U$14.P$4 6.83,75.53 R58.2 6.83,80.01 R56.2 3.71,81.89 3.17,82.42 3.17,87 5.71,89.53 RS485_RX_DATA_LOGGER.6
A_RX_ENERGY_FLOW
  Top 0.203: RS485_RX_ENERGY_FLOW.6 26.19,24.24 25.81,24.62 25.81,26.53 24.16,28.18 22.89,28.18 22.23,28.84 R10.2 19.95,29.96 R17.2 17.4,27.41 17.4,26.8 14.35,23.75 10,23.75 U$7.P$5
A_RX_STEERING_WHEEL
  Top 0.203: R5.2 67.31,33.77 67.67,33.77 R8.2 | U$6.P$2 85.66,17.97
  Top 0.254: RS485_RX_STEERING_WHEEL.6 60.04,40.6 60.15,40.72 61.06,40.72 61.59,40.18 61.59,37.53 R5.2 | U$6.P$2 83.61,17.99 74.93,26.67 74.93,30.45 71.62,33.77 67.31,33.77
A_TX_DATA_LOGGER
  Top 0.203: R44.2 20.05,61.55 R42.2 23.93,61.55 24.92,60.56 24.92,56.63 25.56,55.99 RS485_TX_DATA_LOGGER.6 | 19.46,61.35 R44.2 | R44.2 13.62,61.35 12.12,62.85 U$14.P$3
A_TX_ENERGY_FLOW
  Top 0.203: RS485_TX_ENERGY_FLOW.6 26.07,39.48 25.43,40.12 25.43,42.15 23.65,43.93 22.87,43.93 R24.2 22.05,44.08 R26.2 19.49,44.08 14.15,38.74 14.15,31.75 8.42,26.02 U$7.P$4
A_TX_STEERING_WHEEL
  Top 0.203: 67.75,16.7 R20.2 68.58,16.7 74.07,16.7 79.29,11.48 88.86,11.48 U$6.P$4
  Top 0.254: RS485_TX_STEERING_WHEEL.6 64.08,24.24 65.47,22.85 R19.2 65.88,16.7 68.58,16.7
B_RX_DATA_LOGGER
  Top 0.203: U$14.P$2 10.31,72.92 10.31,78.74 R58.1 8.87,80.19 8.87,82.04 R57.1 6.73,84.18 6.73,87.63 7.37,88.27 RS485_RX_DATA_LOGGER.7
B_RX_ENERGY_FLOW
  Top 0.203: RS485_RX_ENERGY_FLOW.7 25.94,22.97 24.92,23.99 24.92,25.51 23.76,26.68 R11.1 20.18,26.68 R17.1 14.65,21.82 U$7.P$2
B_RX_STEERING_WHEEL
  Top 0.203: R9.1 67.42,36.87 R8.1 71.31,36.56 77.24,30.63 77.24,26.98 84.02,20.19 88.96,20.19 U$6.P$5
  Top 0.254: R9.1 62.59,39.28 62.59,40.91 61.53,41.97 RS485_RX_STEERING_WHEEL.7
B_TX_DATA_LOGGER
  Top 0.203: 19.92,58.43 R43.1 23.63,58.43 24.29,57.77 24.29,55.48 25.05,54.72 RS485_TX_DATA_LOGGER.7 | 19.92,58.43 R44.1 11.6,58.51 6.62,63.49 U$14.P$6 | 19.11,58.43 19.92,58.43
B_TX_ENERGY_FLOW
  Top 0.203: RS485_TX_ENERGY_FLOW.7 25.56,38.21 24.54,39.23 24.54,41.26 23.88,41.92 R25.1 20.53,41.92 R26.1 18.42,41.23 15.25,38.06 15.25,36.77 15.24,36.76 15.24,27.69 U$7.P$1
B_TX_STEERING_WHEEL
  Top 0.203: R21.1 68.23,21.91 R20.1 73.31,19.54 77.77,15.09 84.34,15.09 85.64,13.79 U$6.P$1
  Top 0.254: R21.1 67.86,21.95 64.3,25.51 RS485_TX_STEERING_WHEEL.7
EMERGENCY_BUTTON
  Bottom 0.203: R6.2 27.81,78.44 25.88,78.44 C4.2 25.37,77.93 25.37,76.61 26.8,75.18 26.8,72.26 28.08,70.98 LEFT_GOLDPIN.19
EMERGENCY_RELAY_GPIO  (via drill 0.35)  (1 unrouted)
  Top 0.254: Q8.1 71.22,45.66 R36.1 66.29,45.03 v65.63,44.37
  Bottom 0.305: R51.1 65.1,13.66 RIGHT_GOLDPIN.37 | R51.2 65.1,43.84 v65.63,44.37
EMERGENCY_RELAY_MOSFET
  Top 1.27: Q8.4 84.47,43.38 87.21,40.64 U$4.P$2 87.25,39.33 87.25,34.92 U$3.P$1
GND  (via drill 0.35)
  Top 0.203: RS485_RX_STEERING_WHEEL.2 RS485_RX_STEERING_WHEEL.3 | C2.1 69.07,31.05 C3.1 71.38,31.1 C13.1 | C9.1 C5.1 C6.1 | C10.1 C8.1 C7.1 | C17.1 C19.1 C16.1 | C37.1 C35.1 C33.1 C34.1 C36.1 | C22.1 C21.1 C18.1 C15.1 C20.1 | RS485_RX_DATA_LOGGER.3 RS485_RX_DATA_LOGGER.2 | RS485_RX_ENERGY_FLOW.3 RS485_RX_ENERGY_FLOW.2
  Top 0.254: C12.1 C11.1 C1.1 | Q7.3 70.97,52.33 R32.2 | Q8.3 71.67,41.1 R36.2
  Top 0.305: Q5.3 74.24,63.01 R31.2 | R46.2 31.62,64.44 C38.1
  Top 0.813: TSR_1_2450.2 58.98,88.7 C27.1 | C27.1 62.03,88.68 C28.1 | C27.1 C26.1 | C28.1 C25.1 | C28.1 68.79,88.68 C23.-
  Bottom 0.203: R34.2 C14.1 | C40.1 C41.1
  other vias: 25.4,48.26 19.05,48.26 24.13,46.99 26.92,32.77 17.91,33.02 26.8,29.97 18.29,16.76 22.1,16.38 27.05,17.53 15.11,14.48 11.43,13.59 8.76,14.1 48.51,7.24 63.55,19.99 73.79,20.95 73.84,29.41 60.71,31.75 59.21,34.42 70.51,49.56 63.75,56.39 60.99,55.58 75.56,61.06 72.77,59.44 74.17,58.55 73.91,50.32 82.55,93.6 91.57,92.33 85.47,89.51 67.44,93.98 50.93,84.84 47.5,68.83 64.77,68.71 58.67,65.02 58.67,60.33 43.69,66.17 35.59,3.99 76.4,49.56 70.99,58.55 60.53,86.89 67.18,90.17 68,57.99 64.77,58.55 68.15,56.03 60.88,19.13 34.54,23.62 27.18,26.8 58.42,45.59 57.23,37.24 28.42,3.15 58.55,16.64 62.74,15.37 50.29,6.99 39.24,30.1 37.08,47.88 41.15,47.88 42.29,30.99 47.47,42.8 12.7,3.81 50.29,15.37 85.5,92.48 79.78,85.83 50.42,54.61 50.8,68.33 56.52,68.45 73.15,14.99 73.08,26.11 70.71,62.23 87.58,93.9 90.78,94.69 12.57,39.12 8.76,31.5 13.84,48.01 42.29,17.02 73.15,5.71 66.8,5.71 60.45,5.71 92.2,28.57 89.66,31.11 88.39,26.04 94.74,29.84 74.42,37.47 78.23,34.92 87.12,59.05 92.2,61.59 84.58,8.26 87.12,5.71 36.04,7.59 36.55,5.18 39.09,5.18 40.72,15.34 11.35,9.35 11.66,5.92 14.05,10.59 17.73,12.5 89.66,46.35 75.97,75.67 75.69,33.66 57.4,66.29 57.4,62.48 57.4,59.05 43.94,60.45 46.35,54.23 43.94,57.91 70.36,23.11 74.17,24.13 65.53,47.37 79.78,72.36 66.45,77.83 61.62,79.35 60.48,95.22 58.7,76.81 61.37,77.06 80.54,82.52 41.53,84.58 37.97,82.3 40.77,82.42 41.15,88.65 31.62,83.19 23.11,83.44 25.78,83.44 31.37,90.68 22.1,93.09 13.08,94.61 3.81,90.17 5.59,87.5 10.54,85.22 14.22,77.34 3.05,80.14 15.75,72.39 28.96,68.07 28.83,64.26 8.13,59.31 14.73,64.14 16.76,56.9 9.53,63.5 7.75,55.37 7.24,40.39 11.94,34.42 17.65,36.7 23.75,31.75 10.03,42.55 15.11,44.45 8.64,36.2 3.43,59.82 23.11,75.44 9.27,92.84 15.75,67.31 13.46,56.52 12.19,60.33 25.02,62.99 33.27,92.33 16.38,88.52 50.14,40.64
  pour Top (isolate 0.305, rank 2): -5.08,101.09 -5.08,-6.35 105.41,-6.35 105.41,101.09
  pour Bottom (isolate 0.305): -10.16,109.32 -10.16,-10.16 109.22,-10.16 109.22,109.32
  pour Top (no thermals): 72.09,42.34 72.09,39.85 75.82,39.85 75.82,42.34
  pour Top (no thermals): 72.14,53.57 72.14,51.1 75.92,51.1 75.92,53.57
  pour Top (no thermals): 75.21,64.24 75.21,61.87 78.94,61.87 78.94,64.24
H2_ANALOG  (via drill 0.35)
  Top 0.203: U$9.PIN3 44.4,92.25 v44.4,82.35
  Bottom 0.203: v44.4,82.35 44.4,80.46 R33.2
H2_ANALOG_GPIO  (via drill 0.35)
  Top 0.203: v28.22,75.69 28.22,73.64 LEFT_GOLDPIN.22
  Bottom 0.203: R33.1 R34.1 C14.2 36.47,76.05 28.57,76.05 v28.22,75.69
H2_DIGITAL
  Top 0.203: LEFT_GOLDPIN.18 30.82,70.98 31.9,72.06 31.9,74.55 33.78,76.43 33.78,86.67 39.34,92.23 U$9.PIN1
HORN_GPIO  (via drill 0.35)  (1 unrouted)
  Top 0.305: Q5.1 74.55,67.57 R31.1 72,66.56 v70.63,65.2 v70.63,65.19
  Bottom 0.305: R49.2 68.74,15.39 RIGHT_GOLDPIN.38 | R49.1 67.03,19.94 67.03,60.96 67.03,61.1 67.03,61.59 v70.62,65.19 v70.63,65.19
HORN_MOSFET
  Top 1.016: U$11.P$1 89.62,68.07 U$10.P$2
  Top 3.048: Q5.4 83.94,66.36 | 83.62,65.61 Q5.4 | U$10.P$2 85.23,71.19 83.94,69.9 Q5.4
N$1
  Top 0.203: RS485_RX_ENERGY_FLOW.1 33.94,21.7 34.42,21.22 R28.2 R2.2 37.64,21.23 Q3.3
N$2
  Top 0.203: RS485_RX_ENERGY_FLOW.4 34.6,25.51 R7.2
N$3
  Top 0.203: R18.2 35.57,36.46 35.08,36.94 RS485_TX_ENERGY_FLOW.1
N$4
  Top 0.203: R22.2 37.52,37.83 34.58,37.83 34.2,38.21 RS485_TX_ENERGY_FLOW.2
N$5
  Top 0.203: R23.2 39.05,38.85 35.21,38.85 34.58,39.48 RS485_TX_ENERGY_FLOW.3
N$6
  Top 0.203: RS485_TX_ENERGY_FLOW.4 34.6,40.75 R30.2 35.57,40.75 Q4.3
N$8
  Top 0.508: FUSE_SPEED.1 12.19,53.85 9.75,51.4 9.75,49.01 U$5.P$1
N$9
  Top 0.203: R37.2 35.62,53.73 35.34,53.45 RS485_TX_DATA_LOGGER.1
N$10
  Top 0.203: R40.2 38.89,54.98 38.51,55.36 34.07,55.36 33.43,54.72 RS485_TX_DATA_LOGGER.2
N$11
  Bottom 0.203: R1.2 R6.1 27.69,81.41 27.69,84.92 U$13.P$2
N$12
  Top 0.203: RS485_TX_DATA_LOGGER.3 39.53,55.99 41.43,54.09 R41.2
N$13
  Top 0.203: Q6.3 35.24,57.9 R48.2 34.7,57.36 34.7,57.26 RS485_TX_DATA_LOGGER.4
N$14  (via drill 0.35)
  Top 0.813: v45.21,89.92 45.19,89.94 45.19,90.75 46.71,92.28 U$9.PIN4
  Bottom 0.813: FUSE_H2.2 45.62,89.51 v45.21,89.92
N$15
  Top 0.813: FUSE_STEERING_WHEEL.1 82.8,24.54 85.16,22.19 U$6.P$3
N$16  (via drill 0.35)
  Top 0.254: Q1.3 52.12,36.11 52.12,39.52 v52.98,40.39 52.98,42.27 53.96,43.24 RS485_RX_STEERING_WHEEL.1
  Bottom 0.203: 56.75,44.97 R39.2 55.92,45.42 R3.2
  Bottom 0.254: R3.2 51.71,43.52 51.71,41.66 v52.98,40.39
N$17
  Top 0.254: R4.2 53.85,38.36 54.73,39.24 RS485_RX_STEERING_WHEEL.4
N$18
  Top 0.203: RS485_TX_STEERING_WHEEL.1 55.89,26.78 R14.2
N$19
  Top 0.203: RS485_TX_STEERING_WHEEL.2 54.59,25.51 52.86,27.24 R15.2
N$20
  Top 0.203: RS485_TX_STEERING_WHEEL.3 57.86,24.27 52.84,24.27 50.32,26.78 R16.2
N$21
  Top 0.203: RS485_TX_STEERING_WHEEL.4 56.29,22.97 R13.2 53.02,19.69 Q2.3
N$22
  Top 0.813: FUSE_IN.2 76.69,79.05 DIODE_VIN.C
N$23  (via drill 0.35)
  Top 0.305: Q7.1 71.68,56.89 R32.1 70.23,55.67 v68.66,54.1
  Bottom 0.305: R50.2 68.66,21.06 v68.66,54.1
N$24  (via drill 0.35)
  Top 0.203: v21.79,9.63 21.79,8.74 21.28,8.23 U$8.P$2 22.96,5.94 R53.1
  Bottom 0.203: R52.2 v21.79,9.63
N$25
  Top 0.203: RS485_RX_DATA_LOGGER.1 14.61,87 15.24,86.36 R54.2 R60.2 18.03,84.23 18.03,87.74 Q9.3
N$26
  Top 0.203: RS485_RX_DATA_LOGGER.4 16.15,90.81 R55.2
N$28
  Top 0.203: R35.1 73.46,92.82 LED_PWR.A
N$32
  Top 0.305: TSR_1_2450.1 54.34,84.95 52.89,83.5 52.89,80.58 FUSE_MCU2.1
  Top 0.813: TSR_1_2450.1 60.31,82.4 C26.2 C25.2 68.82,82.4 C23.+ 70.42,80.33 FUSE_IN.1
NUCLEO_RX_DATA_LOGGER  (via drill 0.35)
  Top 0.203: Q9.2 20.52,89.18 R59.2 33.88,89.18 v33.91,89.15 | LEFT_GOLDPIN.16 35.66,70.98 34.67,71.96 34.67,85.72 v35.43,86.49
  Bottom 0.203: v35.43,86.49 35.43,87.63 v33.91,89.15
NUCLEO_RX_ENERGY_FLOW
  Top 0.203: Q3.2 40.59,26.65 41.66,26.65 R27.2 43.44,26.68 44.2,25.92 44.2,21.55 38.77,16.11 32.8,16.11 30.64,13.95 RIGHT_GOLDPIN.23
NUCLEO_RX_STEERING_WHEEL
  Top 0.203: Q1.2 49.54,34.58 R38.2 46.67,36.08 46.67,43.57 71.28,68.18 LEFT_GOLDPIN.2
NUCLEO_TX_DATA_LOGGER  (via drill 0.35)
  Top 0.203: R47.2 40.24,59.83 Q6.2 | R47.2 42.04,60.44 | R47.2 42.67,61.06 v42.67,61.85
  Bottom 0.203: v42.67,61.85 42.67,66.56 LEFT_GOLDPIN.15
NUCLEO_TX_ENERGY_FLOW
  Top 0.203: Q4.2 39.64,41.7 40.62,42.68 R29.2 42.68,42.68 44.91,40.45 44.91,13.78 45.85,12.84 45.85,12.58 RIGHT_GOLDPIN.29
NUCLEO_TX_STEERING_WHEEL
  Top 0.203: Q2.2 49.72,17.82 R12.2 48.37,17.82 45.98,20.2 45.98,44 70.14,68.16 70.14,72.37 LEFT_GOLDPIN.39
P$1
  Top 0.813: U$14.P$1 12.38,75.06 FUSE_DATA_LOGGER.1
RESET_BUTTON
  Top 0.203: R53.2 C39.2 31.11,6.56 30.64,7.03 RIGHT_GOLDPIN.18
SOLENOID_VALVE_GPIO
  Bottom 0.305: R50.1 71.28,15.59 RIGHT_GOLDPIN.39
SOLENOID_VALVE_MOSFET
  Top 1.27: 81.08,54.61 Q7.4 U$1.P$2 88.39,53.43 88.39,48.84 U$2.P$1
SPEED_SENSOR  (via drill 0.35)
  Top 0.203: LEFT_GOLDPIN.21 24.67,73.52 23.4,72.25 23.4,68.58 18.19,63.37 v18.16,63.37
  Bottom 0.203: v18.16,63.37 6.83,52.04 U$5.P$2
V_BATTERY_GPIO
  Top 0.203: LEFT_GOLDPIN.17 34.45,69.71 34.45,67.34 R46.1
  Top 0.305: R46.1 34.59,67.31 34.55,67.27 C38.2 35.69,65.46 R45.1
VIN  (via drill 0.35)
  Top 0.813: v78.99,36.17 82.2,32.97 FUSE_STEERING_WHEEL.2 | FUSE_DATA_LOGGER.2 20.45,75.06 30.48,85.09 v32,85.09
  Top 1.016: U$11.P$2 92.16,71.03 U$10.P$1 | DIODE_VIN.A 79.3,90.92 U$15.P2
  Top 1.27: U$1.P$1 92.71,50.62 91.01,48.92 U$2.P$2 | U$4.P$1 92.71,35.81 U$3.P$2
  Top 3.048: U$10.P$1 90.04,73.15 90.04,80.18 U$15.P2
  Bottom 0.813: v78.99,36.17 78.97,36.17 77.88,37.26 77.88,75.43 83.77,81.32 U$15.P2 | 53.67,91.52 53.66,91.53 51.47,91.53 FUSE_H2.1 | v32,85.09 36.83,85.09 38.1,86.36 48.94,86.36 54.1,91.53
  Bottom 1.016: DIODE_VIN.A 76.08,91.53 54.1,91.53 53.66,91.53
  Bottom 1.27: 82.58,67.79 82.58,74.86 88.9,81.18 U$15.P2 | U$1.P$1 92.71,57.66 82.58,67.79 | 82.58,67.79 82.58,49.5 U$4.P$1

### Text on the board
tNames: H2 | EMERGENCY / BUTTON | GND | GND | VIN | BATTERY | DIGITAL | ANALOG | +5V | SIGNAL | GND | GND | VIN | DATA_LOGGER | A_RX | +12V | HORN | HORN | VIN | GND | B_RX | B_TX | A_TX | GND | VALVE | VALVE | VIN | SPEED_SENSOR | SIGNAL | GND | +5V | GND | GND | EMERGENCY_RELAY | RELAY | VIN | ENERGY_FLOW | A_TX | B_TX | VIN | STEERING_WHEEL | HYDROGREEN TEAM / Author: Alicja Miękina / Date: 08.04.2021 / PCB_Master_0.0.2 | VIN | GND | A_RX | B_RX | A_RX | B_RX | GND | GND | B_TX | A_TX | RESET_BUTTON
bNames: HYDROGREEN TEAM / Author: Alicja Miękina / Date: 08.04.2020 / PCB_Master_0.0.2
tValues: BATTERY | DATA_RECORD | HORN | SPEED_SENSOR | VALVE | USB_CONVERTER | STEERING_WHEEL | ENERGY_FLOW

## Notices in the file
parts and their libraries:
Wurth_Elektronik_Electromechanic_Board_t: Copyright: Würth Elektronik
